FUNCTION "Consensi Linea" : VOID
TITLE =Gestione consensi linea pallet
AUTHOR : MassimoZ
FAMILY : NovaSrl
VERSION : 0.1

BEGIN
NETWORK
TITLE ======== Consensi Vari =======



NETWORK
TITLE =Forzatura dell'Override Limite Max 100%
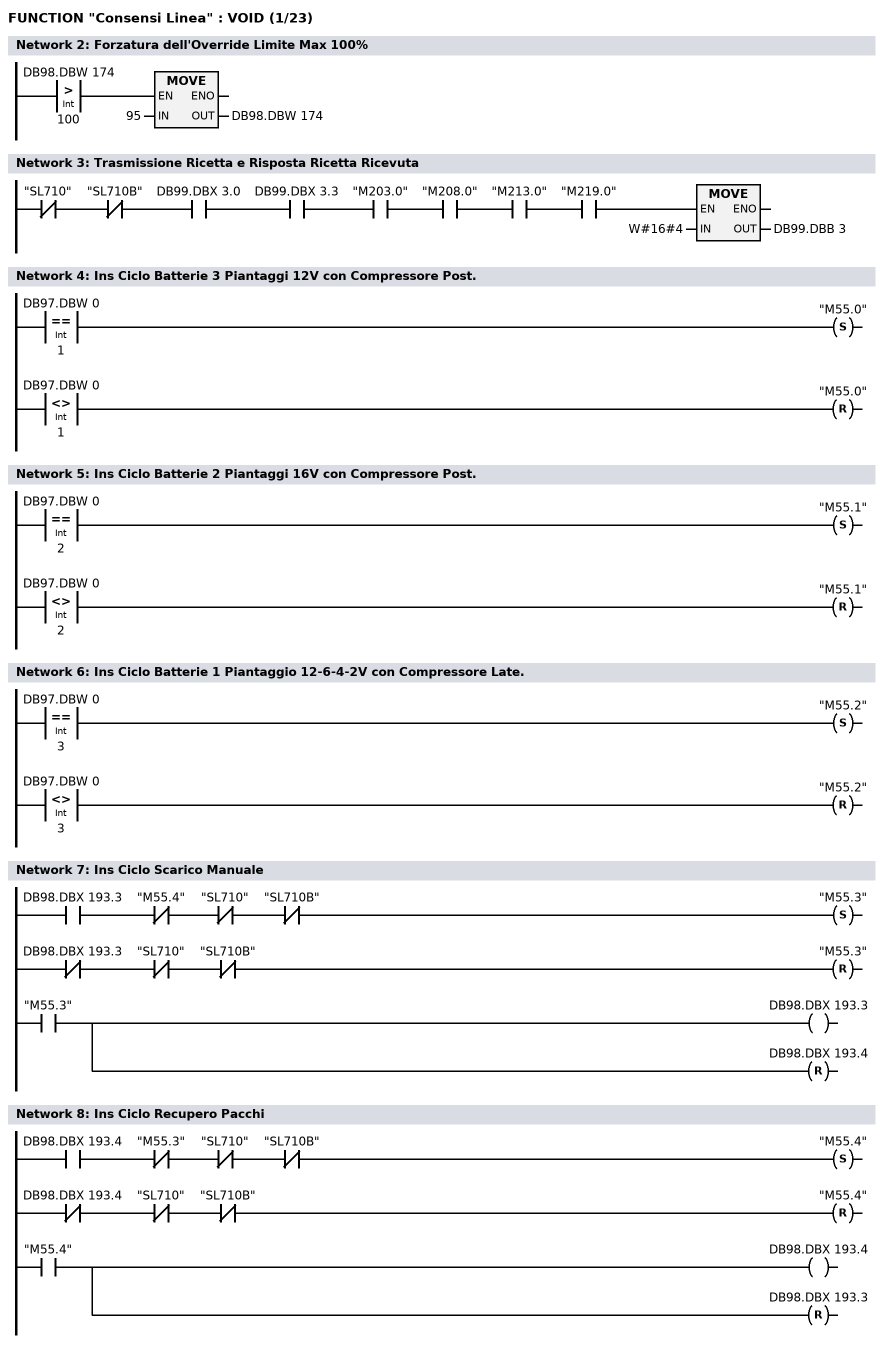
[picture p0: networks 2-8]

      U(    ;
      L     DB98.DBW  174;
      L     100;
      >I    ;
      )     ;
      SPBNB _001;
      L     95;
      T     DB98.DBW  174;
_001: NOP   0;
NETWORK
TITLE =Trasmissione Ricetta e Risposta Ricetta Ricevuta

      UN    "SL710";
      UN    "SL710B";
      U     DB99.DBX    3.0;
      U     DB99.DBX    3.3;
      U     "M203.0";
      U     "M208.0";
      U     "M213.0";
      U     "M219.0";
      SPBNB _002;
      L     W#16#4;
      T     DB99.DBB    3;
_002: NOP   0;
NETWORK
TITLE =Ins Ciclo Batterie 3 Piantaggi 12V con Compressore Post.

      U(    ;
      L     DB97.DBW    0;
      L     1;
      ==I   ;
      )     ;
      S     "M55.0";
      U(    ;
      L     DB97.DBW    0;
      L     1;
      <>I   ;
      )     ;
      R     "M55.0";
      NOP   0;
NETWORK
TITLE =Ins Ciclo Batterie 2 Piantaggi 16V con Compressore Post.

      U(    ;
      L     DB97.DBW    0;
      L     2;
      ==I   ;
      )     ;
      S     "M55.1";
      U(    ;
      L     DB97.DBW    0;
      L     2;
      <>I   ;
      )     ;
      R     "M55.1";
      NOP   0;
NETWORK
TITLE =Ins Ciclo Batterie 1 Piantaggio 12-6-4-2V con Compressore Late.

      U(    ;
      L     DB97.DBW    0;
      L     3;
      ==I   ;
      )     ;
      S     "M55.2";
      U(    ;
      L     DB97.DBW    0;
      L     3;
      <>I   ;
      )     ;
      R     "M55.2";
      NOP   0;
NETWORK
TITLE =Ins Ciclo Scarico Manuale

      U     DB98.DBX  193.3;
      UN    "M55.4";
      UN    "SL710";
      UN    "SL710B";
      S     "M55.3";
      UN    DB98.DBX  193.3;
      UN    "SL710";
      UN    "SL710B";
      R     "M55.3";
      U     "M55.3";
      =     DB98.DBX  193.3;
      R     DB98.DBX  193.4;
NETWORK
TITLE =Ins Ciclo Recupero Pacchi

      U     DB98.DBX  193.4;
      UN    "M55.3";
      UN    "SL710";
      UN    "SL710B";
      S     "M55.4";
      UN    DB98.DBX  193.4;
      UN    "SL710";
      UN    "SL710B";
      R     "M55.4";
      U     "M55.4";
      =     DB98.DBX  193.4;
      R     DB98.DBX  193.3;
NETWORK
TITLE =Visualizzazione a Pannello del Ciclo 3 Piantaggi Inserito
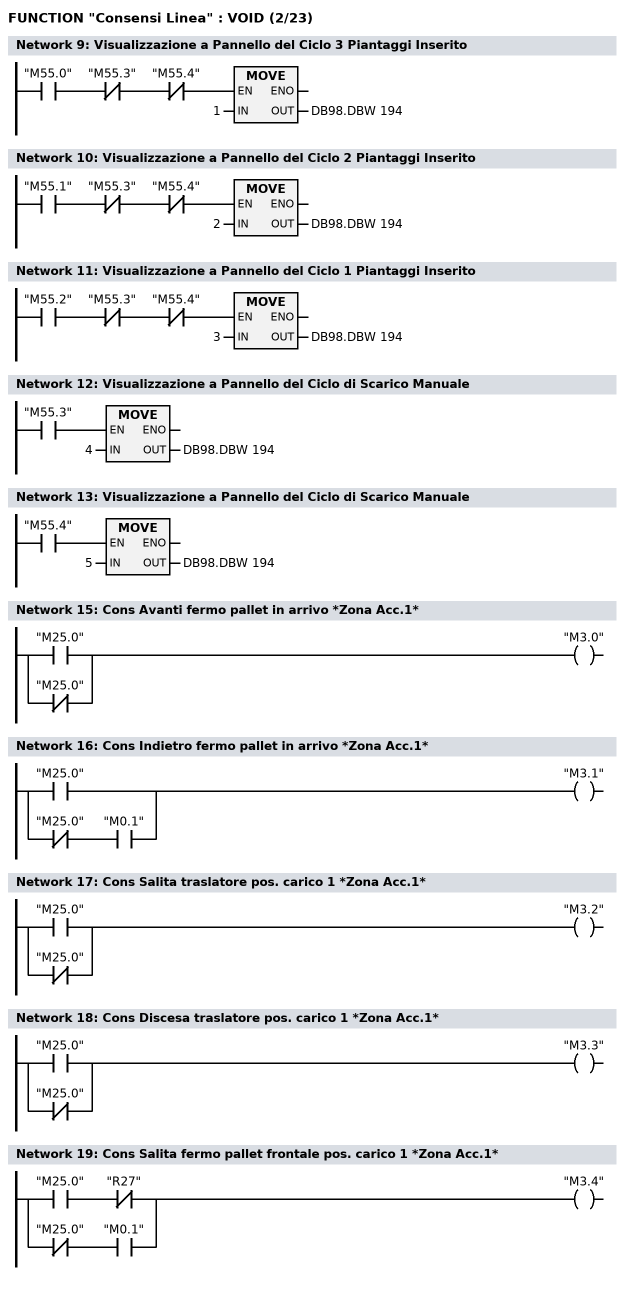
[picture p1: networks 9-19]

      U     "M55.0";
      UN    "M55.3";
      UN    "M55.4";
      SPBNB _003;
      L     1;
      T     DB98.DBW  194;
_003: NOP   0;
NETWORK
TITLE =Visualizzazione a Pannello del Ciclo 2 Piantaggi Inserito

      U     "M55.1";
      UN    "M55.3";
      UN    "M55.4";
      SPBNB _004;
      L     2;
      T     DB98.DBW  194;
_004: NOP   0;
NETWORK
TITLE =Visualizzazione a Pannello del Ciclo 1 Piantaggi Inserito

      U     "M55.2";
      UN    "M55.3";
      UN    "M55.4";
      SPBNB _005;
      L     3;
      T     DB98.DBW  194;
_005: NOP   0;
NETWORK
TITLE =Visualizzazione a Pannello del Ciclo di Scarico Manuale

      U     "M55.3";
      SPBNB _006;
      L     4;
      T     DB98.DBW  194;
_006: NOP   0;
NETWORK
TITLE =Visualizzazione a Pannello del Ciclo di Scarico Manuale

      U     "M55.4";
      SPBNB _007;
      L     5;
      T     DB98.DBW  194;
_007: NOP   0;
NETWORK
TITLE ========= Consensi Zona Accatastatrice 1 =======



NETWORK
TITLE =Cons Avanti fermo pallet in arrivo *Zona Acc.1*

      O     "M25.0";
      ON    "M25.0";
      =     "M3.0";
NETWORK
TITLE =Cons Indietro fermo pallet in arrivo *Zona Acc.1*

      O     "M25.0";
      O     ;
      UN    "M25.0";
      U     "M0.1";
      =     "M3.1";
NETWORK
TITLE =Cons Salita traslatore pos. carico 1 *Zona Acc.1*

      O     "M25.0";
      ON    "M25.0";
      =     "M3.2";
NETWORK
TITLE =Cons Discesa traslatore pos. carico 1 *Zona Acc.1*

      O     "M25.0";
      ON    "M25.0";
      =     "M3.3";
NETWORK
TITLE =Cons Salita fermo pallet frontale pos. carico 1 *Zona Acc.1*

      U     "M25.0";
      UN    "R27";
      O     ;
      UN    "M25.0";
      U     "M0.1";
      =     "M3.4";
NETWORK
TITLE =Cons Discesa fermo pallet frontale pos. carico 1 *Zona Acc.1*
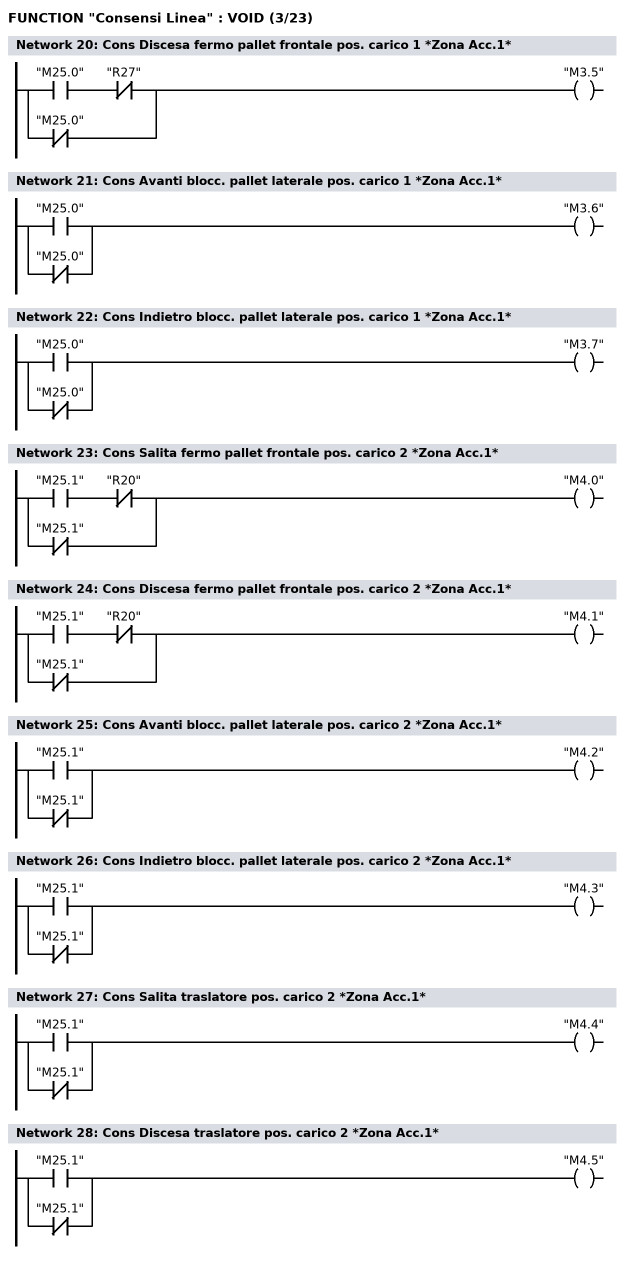
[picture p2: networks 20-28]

      U     "M25.0";
      UN    "R27";
      ON    "M25.0";
      =     "M3.5";
NETWORK
TITLE =Cons Avanti blocc. pallet laterale pos. carico 1 *Zona Acc.1*

      O     "M25.0";
      ON    "M25.0";
      =     "M3.6";
NETWORK
TITLE =Cons Indietro blocc. pallet laterale pos. carico 1 *Zona Acc.1*

      O     "M25.0";
      ON    "M25.0";
      =     "M3.7";
NETWORK
TITLE =Cons Salita fermo pallet frontale pos. carico 2 *Zona Acc.1*

      U     "M25.1";
      UN    "R20";
      ON    "M25.1";
      =     "M4.0";
NETWORK
TITLE =Cons Discesa fermo pallet frontale pos. carico 2 *Zona Acc.1*

      U     "M25.1";
      UN    "R20";
      ON    "M25.1";
      =     "M4.1";
NETWORK
TITLE =Cons Avanti blocc. pallet laterale pos. carico 2 *Zona Acc.1*

      O     "M25.1";
      ON    "M25.1";
      =     "M4.2";
NETWORK
TITLE =Cons Indietro blocc. pallet laterale pos. carico 2 *Zona Acc.1*

      O     "M25.1";
      ON    "M25.1";
      =     "M4.3";
NETWORK
TITLE =Cons Salita traslatore pos. carico 2 *Zona Acc.1*

      O     "M25.1";
      ON    "M25.1";
      =     "M4.4";
NETWORK
TITLE =Cons Discesa traslatore pos. carico 2 *Zona Acc.1*

      O     "M25.1";
      ON    "M25.1";
      =     "M4.5";
NETWORK
TITLE =Cons Salita fermo pallet in uscita *Zona Acc.1*
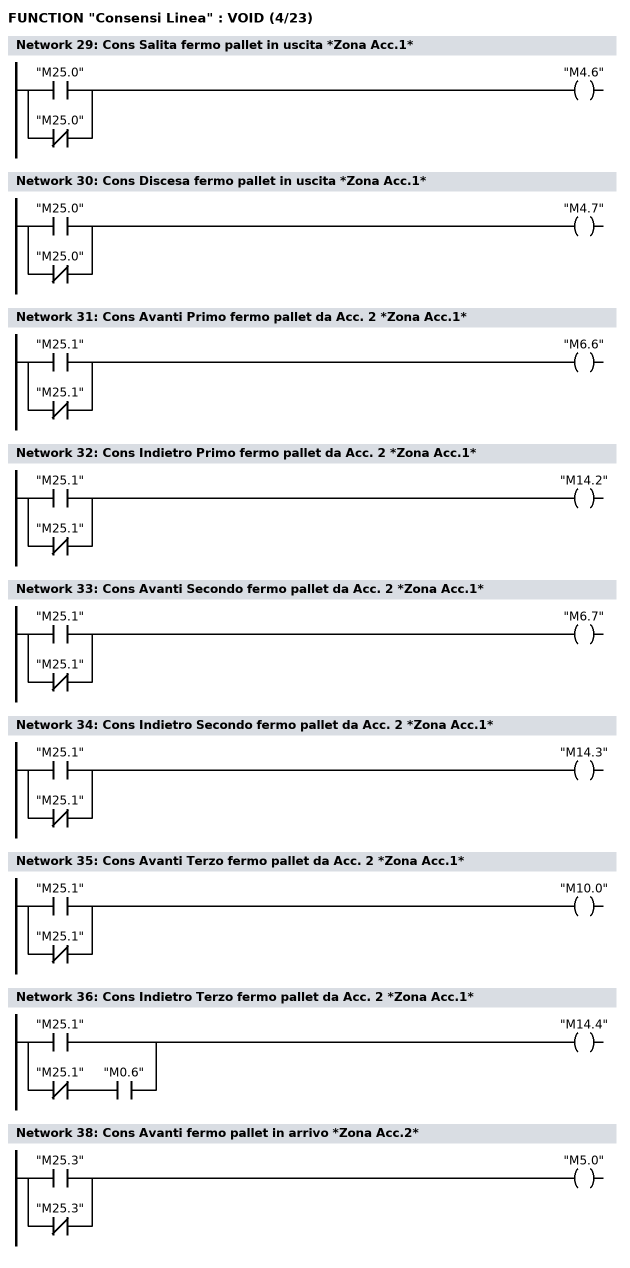
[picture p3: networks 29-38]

      O     "M25.0";
      ON    "M25.0";
      =     "M4.6";
NETWORK
TITLE =Cons Discesa fermo pallet in uscita *Zona Acc.1*

      O     "M25.0";
      ON    "M25.0";
      =     "M4.7";
NETWORK
TITLE =Cons Avanti Primo fermo pallet da Acc. 2 *Zona Acc.1*

      O     "M25.1";
      ON    "M25.1";
      =     "M6.6";
NETWORK
TITLE =Cons Indietro Primo fermo pallet da Acc. 2 *Zona Acc.1*

      O     "M25.1";
      ON    "M25.1";
      =     "M14.2";
NETWORK
TITLE =Cons Avanti Secondo fermo pallet da Acc. 2 *Zona Acc.1*

      O     "M25.1";
      ON    "M25.1";
      =     "M6.7";
NETWORK
TITLE =Cons Indietro Secondo fermo pallet da Acc. 2 *Zona Acc.1*

      O     "M25.1";
      ON    "M25.1";
      =     "M14.3";
NETWORK
TITLE =Cons Avanti Terzo fermo pallet da Acc. 2 *Zona Acc.1*

      O     "M25.1";
      ON    "M25.1";
      =     "M10.0";
NETWORK
TITLE =Cons Indietro Terzo fermo pallet da Acc. 2 *Zona Acc.1*

      O     "M25.1";
      O     ;
      UN    "M25.1";
      U     "M0.6";
      =     "M14.4";
NETWORK
TITLE ========= Consensi Zona Accatastatrice 2 =======



NETWORK
TITLE =Cons Avanti fermo pallet in arrivo *Zona Acc.2*

      O     "M25.3";
      ON    "M25.3";
      =     "M5.0";
NETWORK
TITLE =Cons Indietro fermo pallet in arrivo *Zona Acc.2*
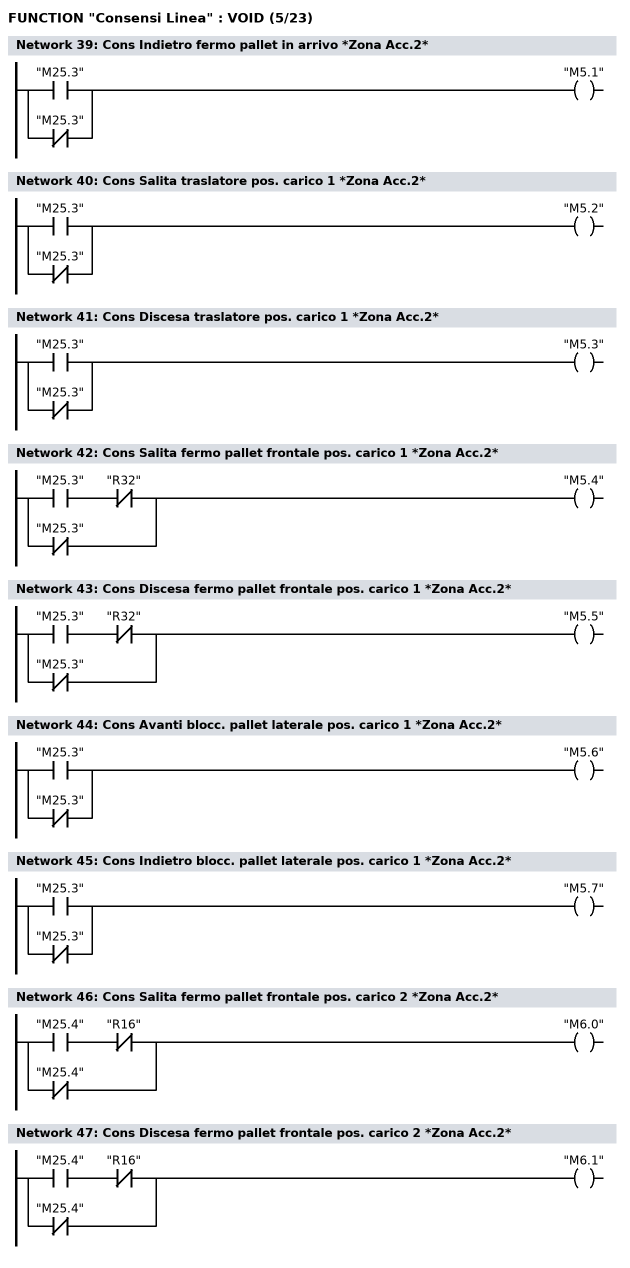
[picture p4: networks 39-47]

      O     "M25.3";
      ON    "M25.3";
      =     "M5.1";
NETWORK
TITLE =Cons Salita traslatore pos. carico 1 *Zona Acc.2*

      O     "M25.3";
      ON    "M25.3";
      =     "M5.2";
NETWORK
TITLE =Cons Discesa traslatore pos. carico 1 *Zona Acc.2*

      O     "M25.3";
      ON    "M25.3";
      =     "M5.3";
NETWORK
TITLE =Cons Salita fermo pallet frontale pos. carico 1 *Zona Acc.2*

      U     "M25.3";
      UN    "R32";
      ON    "M25.3";
      =     "M5.4";
NETWORK
TITLE =Cons Discesa fermo pallet frontale pos. carico 1 *Zona Acc.2*

      U     "M25.3";
      UN    "R32";
      ON    "M25.3";
      =     "M5.5";
NETWORK
TITLE =Cons Avanti blocc. pallet laterale pos. carico 1 *Zona Acc.2*

      O     "M25.3";
      ON    "M25.3";
      =     "M5.6";
NETWORK
TITLE =Cons Indietro blocc. pallet laterale pos. carico 1 *Zona Acc.2*

      O     "M25.3";
      ON    "M25.3";
      =     "M5.7";
NETWORK
TITLE =Cons Salita fermo pallet frontale pos. carico 2 *Zona Acc.2*

      U     "M25.4";
      UN    "R16";
      ON    "M25.4";
      =     "M6.0";
NETWORK
TITLE =Cons Discesa fermo pallet frontale pos. carico 2 *Zona Acc.2*

      U     "M25.4";
      UN    "R16";
      ON    "M25.4";
      =     "M6.1";
NETWORK
TITLE =Cons Avanti blocc. pallet laterale pos. carico 2 *Zona Acc.2*
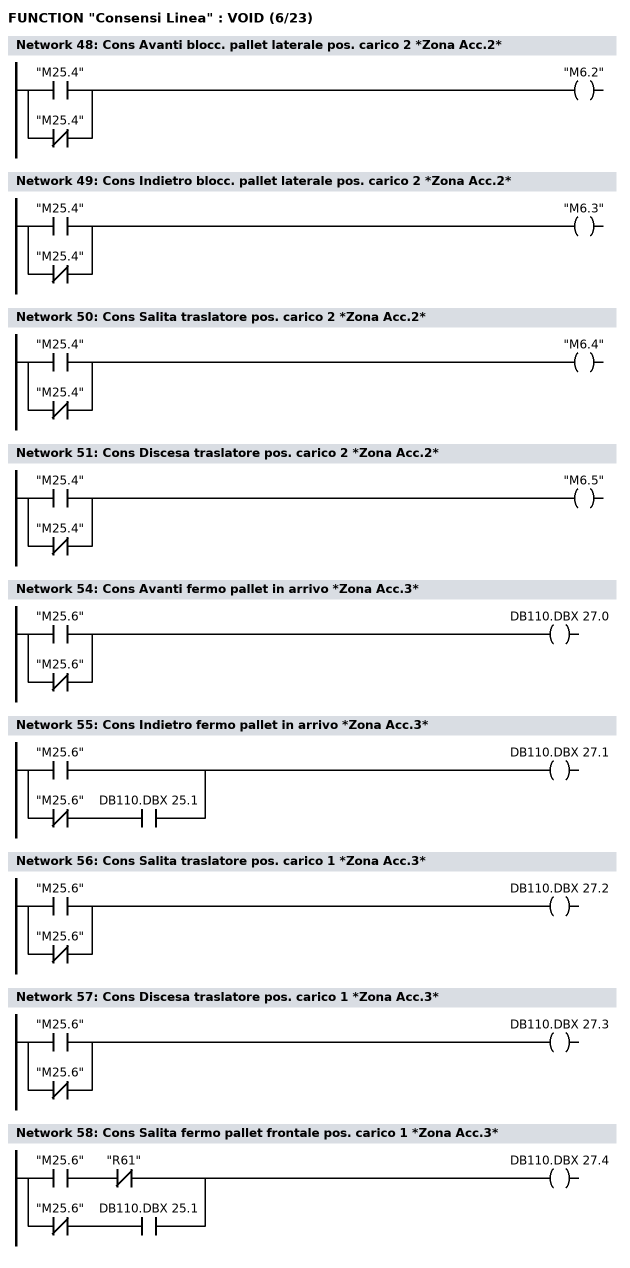
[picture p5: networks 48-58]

      O     "M25.4";
      ON    "M25.4";
      =     "M6.2";
NETWORK
TITLE =Cons Indietro blocc. pallet laterale pos. carico 2 *Zona Acc.2*

      O     "M25.4";
      ON    "M25.4";
      =     "M6.3";
NETWORK
TITLE =Cons Salita traslatore pos. carico 2 *Zona Acc.2*

      O     "M25.4";
      ON    "M25.4";
      =     "M6.4";
NETWORK
TITLE =Cons Discesa traslatore pos. carico 2 *Zona Acc.2*

      O     "M25.4";
      ON    "M25.4";
      =     "M6.5";
NETWORK
TITLE =

NETWORK
TITLE ========= Consensi Zona Accatastatrice 3 =======

NETWORK
TITLE =Cons Avanti fermo pallet in arrivo *Zona Acc.3*

      O     "M25.6";
      ON    "M25.6";
      =     DB110.DBX   27.0;
NETWORK
TITLE =Cons Indietro fermo pallet in arrivo *Zona Acc.3*

      O     "M25.6";
      O     ;
      UN    "M25.6";
      U     DB110.DBX   25.1;
      =     DB110.DBX   27.1;
NETWORK
TITLE =Cons Salita traslatore pos. carico 1 *Zona Acc.3*

      O     "M25.6";
      ON    "M25.6";
      =     DB110.DBX   27.2;
NETWORK
TITLE =Cons Discesa traslatore pos. carico 1 *Zona Acc.3*

      O     "M25.6";
      ON    "M25.6";
      =     DB110.DBX   27.3;
NETWORK
TITLE =Cons Salita fermo pallet frontale pos. carico 1 *Zona Acc.3*

      U     "M25.6";
      UN    "R61";
      O     ;
      UN    "M25.6";
      U     DB110.DBX   25.1;
      =     DB110.DBX   27.4;
NETWORK
TITLE =Cons Discesa fermo pallet frontale pos. carico 1 *Zona Acc.3*
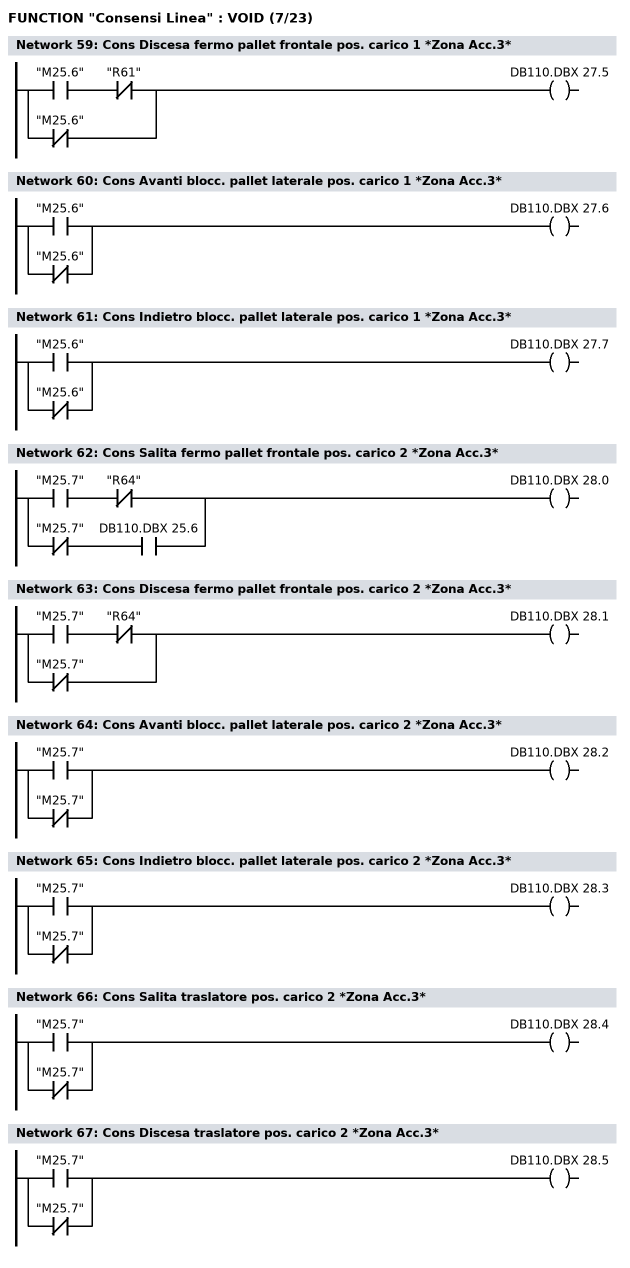
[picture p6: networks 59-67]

      U     "M25.6";
      UN    "R61";
      ON    "M25.6";
      =     DB110.DBX   27.5;
NETWORK
TITLE =Cons Avanti blocc. pallet laterale pos. carico 1 *Zona Acc.3*

      O     "M25.6";
      ON    "M25.6";
      =     DB110.DBX   27.6;
NETWORK
TITLE =Cons Indietro blocc. pallet laterale pos. carico 1 *Zona Acc.3*

      O     "M25.6";
      ON    "M25.6";
      =     DB110.DBX   27.7;
NETWORK
TITLE =Cons Salita fermo pallet frontale pos. carico 2 *Zona Acc.3*

      U     "M25.7";
      UN    "R64";
      O     ;
      UN    "M25.7";
      U     DB110.DBX   25.6;
      =     DB110.DBX   28.0;
NETWORK
TITLE =Cons Discesa fermo pallet frontale pos. carico 2 *Zona Acc.3*

      U     "M25.7";
      UN    "R64";
      ON    "M25.7";
      =     DB110.DBX   28.1;
NETWORK
TITLE =Cons Avanti blocc. pallet laterale pos. carico 2 *Zona Acc.3*

      O     "M25.7";
      ON    "M25.7";
      =     DB110.DBX   28.2;
NETWORK
TITLE =Cons Indietro blocc. pallet laterale pos. carico 2 *Zona Acc.3*

      O     "M25.7";
      ON    "M25.7";
      =     DB110.DBX   28.3;
NETWORK
TITLE =Cons Salita traslatore pos. carico 2 *Zona Acc.3*

      O     "M25.7";
      ON    "M25.7";
      =     DB110.DBX   28.4;
NETWORK
TITLE =Cons Discesa traslatore pos. carico 2 *Zona Acc.3*

      O     "M25.7";
      ON    "M25.7";
      =     DB110.DBX   28.5;
NETWORK
TITLE =Cons Salita fermo pallet in uscita *Zona Acc.3*
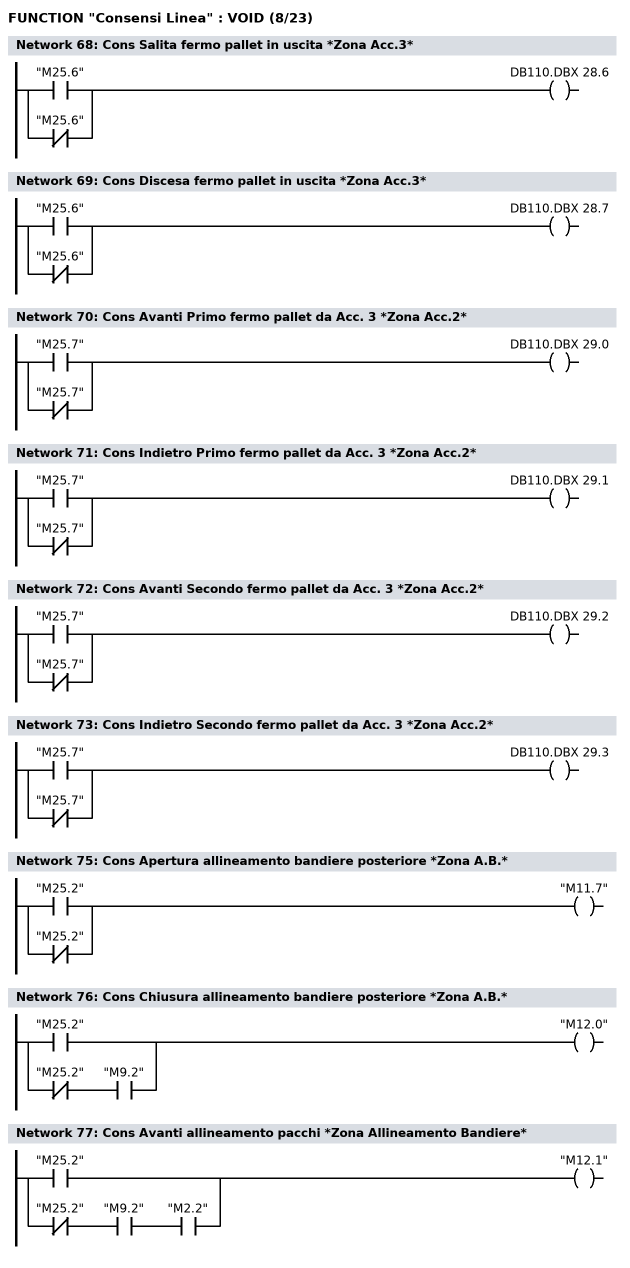
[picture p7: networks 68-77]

      O     "M25.6";
      ON    "M25.6";
      =     DB110.DBX   28.6;
NETWORK
TITLE =Cons Discesa fermo pallet in uscita *Zona Acc.3*

      O     "M25.6";
      ON    "M25.6";
      =     DB110.DBX   28.7;
NETWORK
TITLE =Cons Avanti Primo fermo pallet da Acc. 3 *Zona Acc.2*

      O     "M25.7";
      ON    "M25.7";
      =     DB110.DBX   29.0;
NETWORK
TITLE =Cons Indietro Primo fermo pallet da Acc. 3 *Zona Acc.2*

      O     "M25.7";
      ON    "M25.7";
      =     DB110.DBX   29.1;
NETWORK
TITLE =Cons Avanti Secondo fermo pallet da Acc. 3 *Zona Acc.2*

      O     "M25.7";
      ON    "M25.7";
      =     DB110.DBX   29.2;
NETWORK
TITLE =Cons Indietro Secondo fermo pallet da Acc. 3 *Zona Acc.2*

      O     "M25.7";
      ON    "M25.7";
      =     DB110.DBX   29.3;
NETWORK
TITLE ======== Consensi Zona Allineamento Bandiere =======



NETWORK
TITLE =Cons Apertura allineamento bandiere posteriore *Zona A.B.*

      O     "M25.2";
      ON    "M25.2";
      =     "M11.7";
NETWORK
TITLE =Cons Chiusura allineamento bandiere posteriore *Zona A.B.*

      O     "M25.2";
      O     ;
      UN    "M25.2";
      U     "M9.2";
      =     "M12.0";
NETWORK
TITLE =Cons Avanti allineamento pacchi *Zona Allineamento Bandiere*

      O     "M25.2";
      O     ;
      UN    "M25.2";
      U     "M9.2";
      U     "M2.2";
      =     "M12.1";
NETWORK
TITLE =Cons Indietro allineamento pacchi *Zona Allineamento Bandiere*
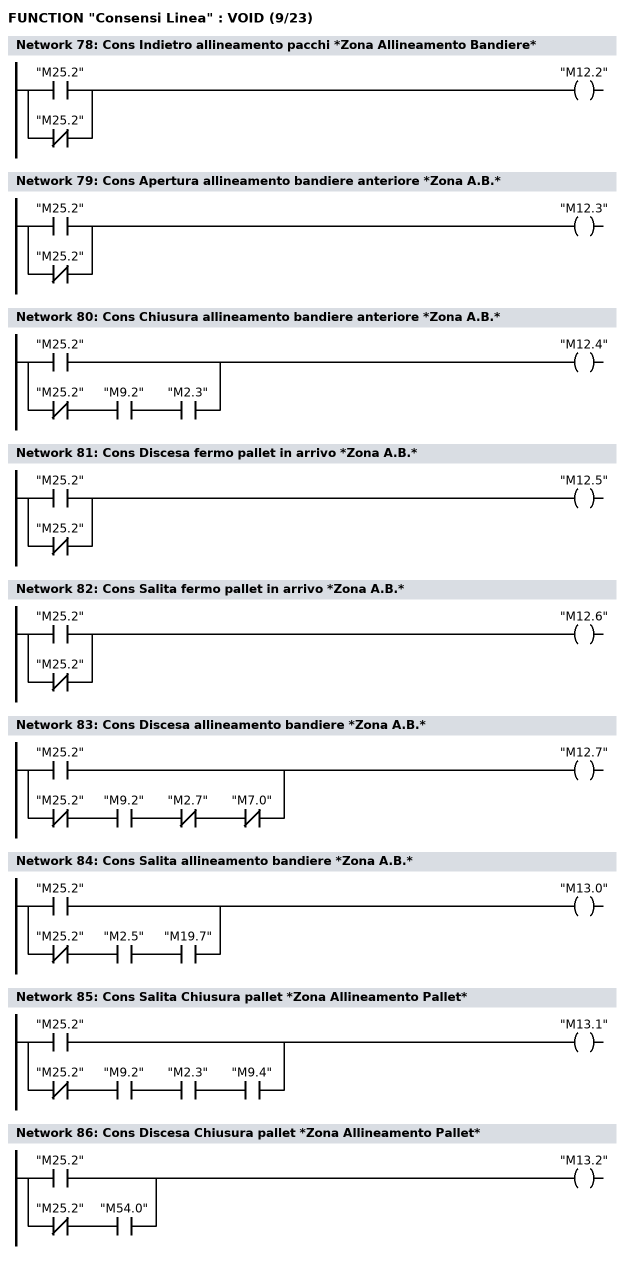
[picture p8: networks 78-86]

      O     "M25.2";
      ON    "M25.2";
      =     "M12.2";
NETWORK
TITLE =Cons Apertura allineamento bandiere anteriore *Zona A.B.*

      O     "M25.2";
      ON    "M25.2";
      =     "M12.3";
NETWORK
TITLE =Cons Chiusura allineamento bandiere anteriore *Zona A.B.*

      O     "M25.2";
      O     ;
      UN    "M25.2";
      U     "M9.2";
      U     "M2.3";
      =     "M12.4";
NETWORK
TITLE =Cons Discesa fermo pallet in arrivo *Zona A.B.*

      O     "M25.2";
      ON    "M25.2";
      =     "M12.5";
NETWORK
TITLE =Cons Salita fermo pallet in arrivo *Zona A.B.*

      O     "M25.2";
      ON    "M25.2";
      =     "M12.6";
NETWORK
TITLE =Cons Discesa allineamento bandiere *Zona A.B.*

      O     "M25.2";
      O     ;
      UN    "M25.2";
      U     "M9.2";
      UN    "M2.7";
      UN    "M7.0";
      =     "M12.7";
NETWORK
TITLE =Cons Salita allineamento bandiere *Zona A.B.*

      O     "M25.2";
      O     ;
      UN    "M25.2";
      U     "M2.5";
      U     "M19.7";
      =     "M13.0";
NETWORK
TITLE =Cons Salita Chiusura pallet *Zona Allineamento Pallet*

      O     "M25.2";
      O     ;
      UN    "M25.2";
      U     "M9.2";
      U     "M2.3";
      U     "M9.4";
      =     "M13.1";
NETWORK
TITLE =Cons Discesa Chiusura pallet *Zona Allineamento Pallet*

      O     "M25.2";
      O     ;
      UN    "M25.2";
      U     "M54.0";
      =     "M13.2";
NETWORK
TITLE =Cons Avanti Chiusura pallet *Zona Allineamento Pallet*
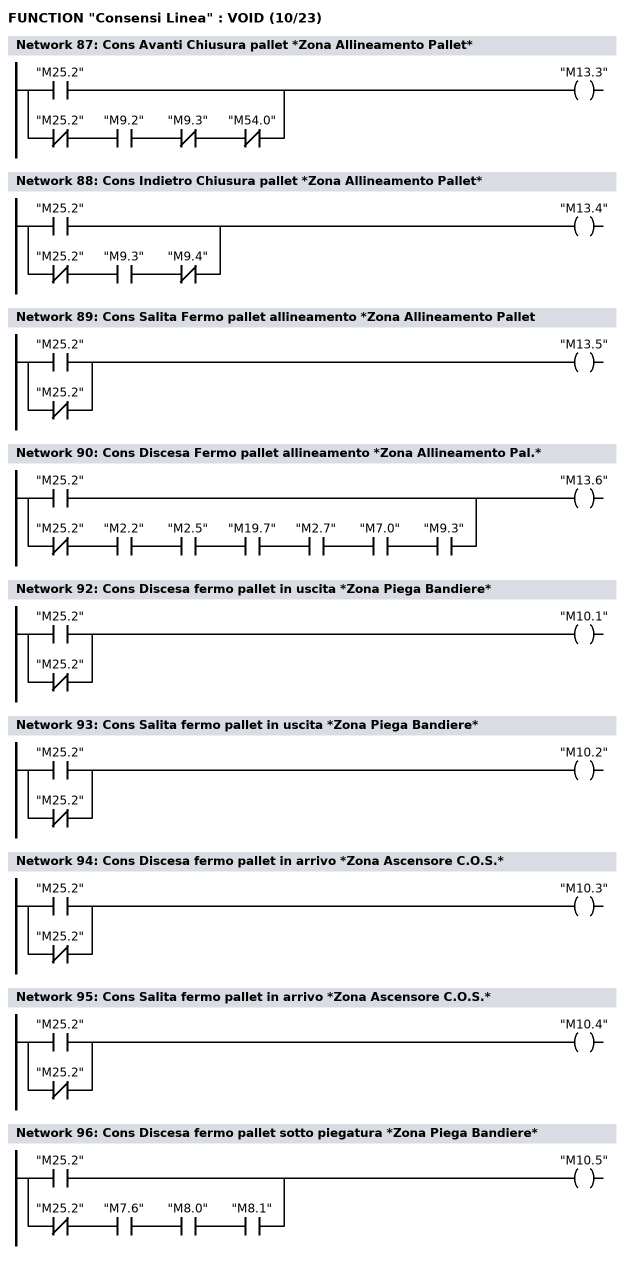
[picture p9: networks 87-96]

      O     "M25.2";
      O     ;
      UN    "M25.2";
      U     "M9.2";
      UN    "M9.3";
      UN    "M54.0";
      =     "M13.3";
NETWORK
TITLE =Cons Indietro Chiusura pallet *Zona Allineamento Pallet*

      O     "M25.2";
      O     ;
      UN    "M25.2";
      U     "M9.3";
      UN    "M9.4";
      =     "M13.4";
NETWORK
TITLE =Cons Salita Fermo pallet allineamento *Zona Allineamento Pallet

      O     "M25.2";
      ON    "M25.2";
      =     "M13.5";
NETWORK
TITLE =Cons Discesa Fermo pallet allineamento *Zona Allineamento Pal.*

      O     "M25.2";
      O     ;
      UN    "M25.2";
      U     "M2.2";
      U     "M2.5";
      U     "M19.7";
      U     "M2.7";
      U     "M7.0";
      U     "M9.3";
      =     "M13.6";
NETWORK
TITLE ======== Consensi Zona Piegatura Bandiere =======



NETWORK
TITLE =Cons Discesa fermo pallet in uscita *Zona Piega Bandiere*

      O     "M25.2";
      ON    "M25.2";
      =     "M10.1";
NETWORK
TITLE =Cons Salita fermo pallet in uscita *Zona Piega Bandiere*

      O     "M25.2";
      ON    "M25.2";
      =     "M10.2";
NETWORK
TITLE =Cons Discesa fermo pallet in arrivo *Zona Ascensore C.O.S.*

      O     "M25.2";
      ON    "M25.2";
      =     "M10.3";
NETWORK
TITLE =Cons Salita fermo pallet in arrivo *Zona Ascensore C.O.S.*

      O     "M25.2";
      ON    "M25.2";
      =     "M10.4";
NETWORK
TITLE =Cons Discesa fermo pallet sotto piegatura *Zona Piega Bandiere*

      O     "M25.2";
      O     ;
      UN    "M25.2";
      U     "M7.6";
      U     "M8.0";
      U     "M8.1";
      =     "M10.5";
NETWORK
TITLE =Cons Salita fermo pallet sotto piegatura *Zona Piega Bandiere*
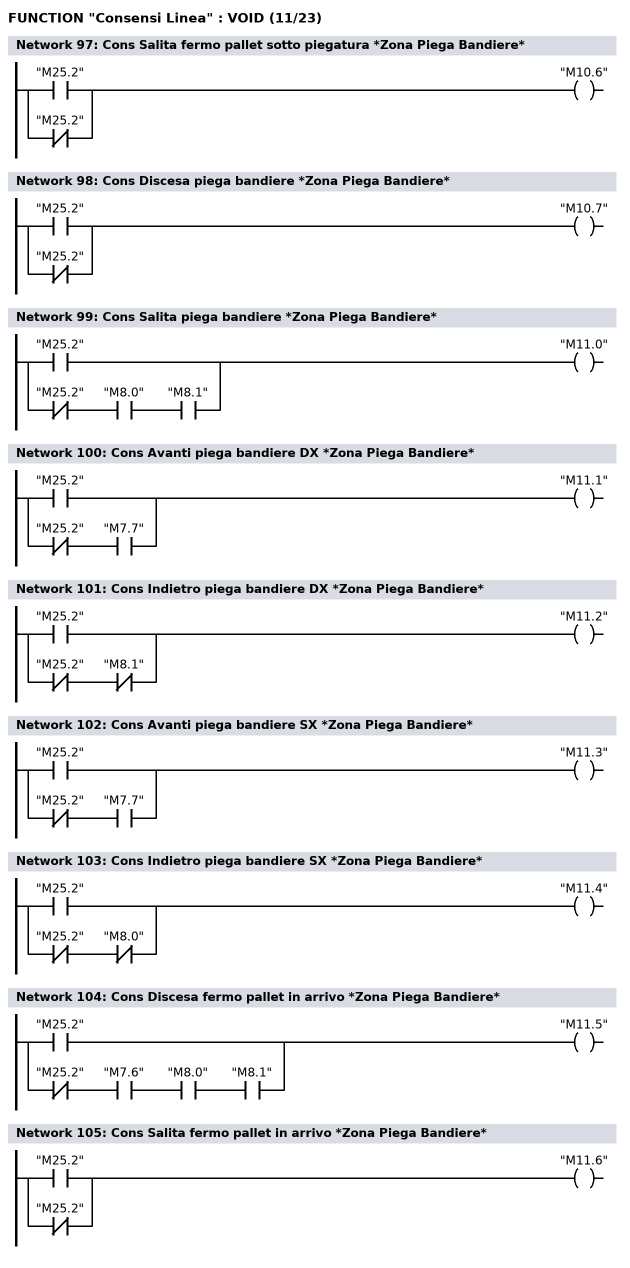
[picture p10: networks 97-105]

      O     "M25.2";
      ON    "M25.2";
      =     "M10.6";
NETWORK
TITLE =Cons Discesa piega bandiere *Zona Piega Bandiere*

      O     "M25.2";
      ON    "M25.2";
      =     "M10.7";
NETWORK
TITLE =Cons Salita piega bandiere *Zona Piega Bandiere*

      O     "M25.2";
      O     ;
      UN    "M25.2";
      U     "M8.0";
      U     "M8.1";
      =     "M11.0";
NETWORK
TITLE =Cons Avanti piega bandiere DX *Zona Piega Bandiere*

      O     "M25.2";
      O     ;
      UN    "M25.2";
      U     "M7.7";
      =     "M11.1";
NETWORK
TITLE =Cons Indietro piega bandiere DX *Zona Piega Bandiere*

      O     "M25.2";
      O     ;
      UN    "M25.2";
      UN    "M8.1";
      =     "M11.2";
NETWORK
TITLE =Cons Avanti piega bandiere SX *Zona Piega Bandiere*

      O     "M25.2";
      O     ;
      UN    "M25.2";
      U     "M7.7";
      =     "M11.3";
NETWORK
TITLE =Cons Indietro piega bandiere SX *Zona Piega Bandiere*

      O     "M25.2";
      O     ;
      UN    "M25.2";
      UN    "M8.0";
      =     "M11.4";
NETWORK
TITLE =Cons Discesa fermo pallet in arrivo *Zona Piega Bandiere*

      O     "M25.2";
      O     ;
      UN    "M25.2";
      U     "M7.6";
      U     "M8.0";
      U     "M8.1";
      =     "M11.5";
NETWORK
TITLE =Cons Salita fermo pallet in arrivo *Zona Piega Bandiere*

      O     "M25.2";
      ON    "M25.2";
      =     "M11.6";
NETWORK
TITLE =Cons Salita Fermo Pallet Anteriore su Ascensore C.O.S.
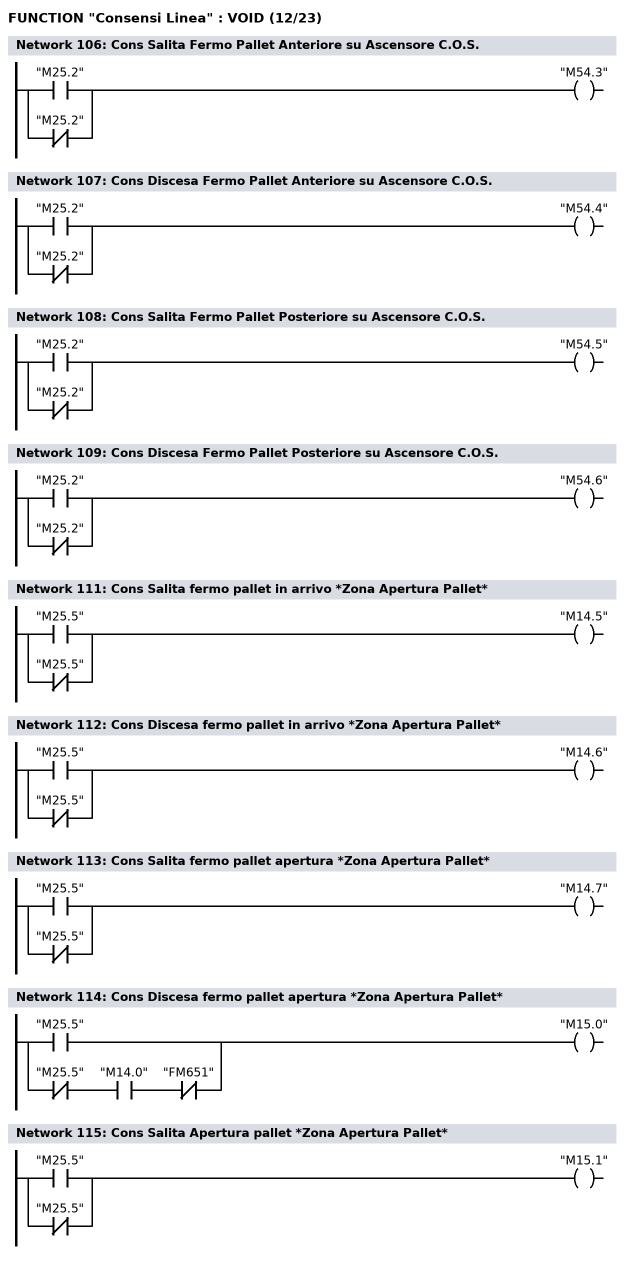
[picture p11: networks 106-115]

      O     "M25.2";
      ON    "M25.2";
      =     "M54.3";
NETWORK
TITLE =Cons Discesa Fermo Pallet Anteriore su Ascensore C.O.S.

      O     "M25.2";
      ON    "M25.2";
      =     "M54.4";
NETWORK
TITLE =Cons Salita Fermo Pallet Posteriore su Ascensore C.O.S.

      O     "M25.2";
      ON    "M25.2";
      =     "M54.5";
NETWORK
TITLE =Cons Discesa Fermo Pallet Posteriore su Ascensore C.O.S.

      O     "M25.2";
      ON    "M25.2";
      =     "M54.6";
NETWORK
TITLE ========= Consensi Zona Apertura Pallet =======



NETWORK
TITLE =Cons Salita fermo pallet in arrivo *Zona Apertura Pallet*

      O     "M25.5";
      ON    "M25.5";
      =     "M14.5";
NETWORK
TITLE =Cons Discesa fermo pallet in arrivo *Zona Apertura Pallet*

      O     "M25.5";
      ON    "M25.5";
      =     "M14.6";
NETWORK
TITLE =Cons Salita fermo pallet apertura *Zona Apertura Pallet*

      O     "M25.5";
      ON    "M25.5";
      =     "M14.7";
NETWORK
TITLE =Cons Discesa fermo pallet apertura *Zona Apertura Pallet*

      O     "M25.5";
      O     ;
      UN    "M25.5";
      U     "M14.0";
      UN    "FM651";
      =     "M15.0";
NETWORK
TITLE =Cons Salita Apertura pallet *Zona Apertura Pallet*

      O     "M25.5";
      ON    "M25.5";
      =     "M15.1";
NETWORK
TITLE =Cons Discesa Apertura pallet *Zona Apertura Pallet*
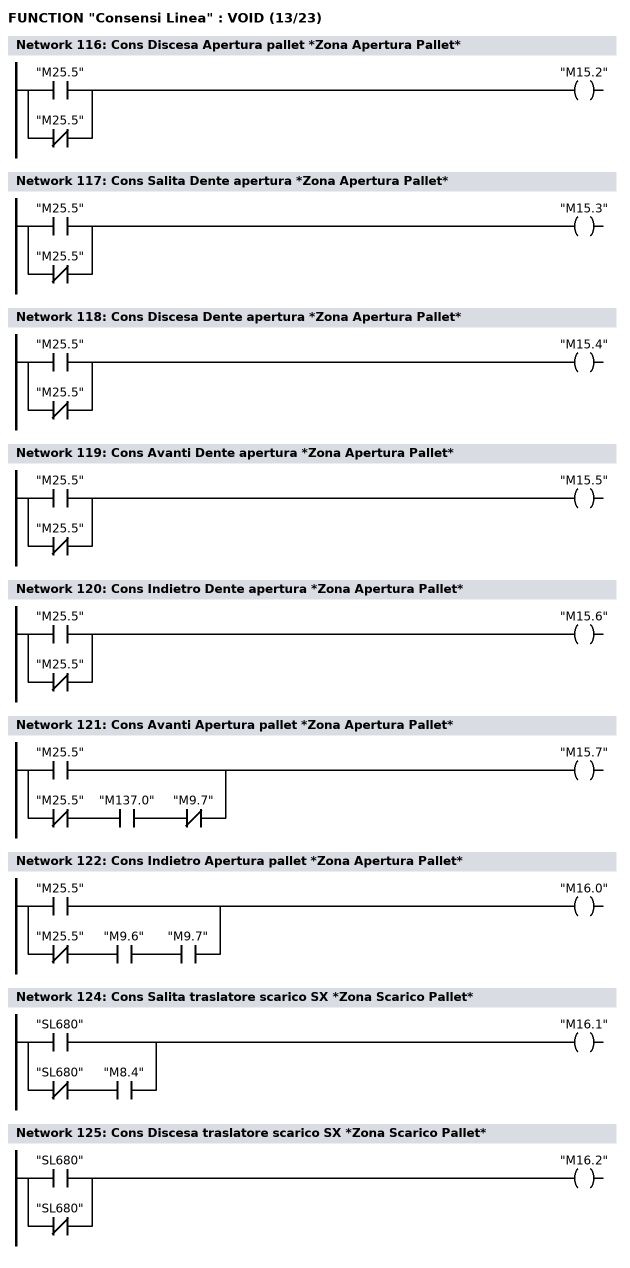
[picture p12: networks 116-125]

      O     "M25.5";
      ON    "M25.5";
      =     "M15.2";
NETWORK
TITLE =Cons Salita Dente apertura *Zona Apertura Pallet*

      O     "M25.5";
      ON    "M25.5";
      =     "M15.3";
NETWORK
TITLE =Cons Discesa Dente apertura *Zona Apertura Pallet*

      O     "M25.5";
      ON    "M25.5";
      =     "M15.4";
NETWORK
TITLE =Cons Avanti Dente apertura *Zona Apertura Pallet*

      O     "M25.5";
      ON    "M25.5";
      =     "M15.5";
NETWORK
TITLE =Cons Indietro Dente apertura *Zona Apertura Pallet*

      O     "M25.5";
      ON    "M25.5";
      =     "M15.6";
NETWORK
TITLE =Cons Avanti Apertura pallet *Zona Apertura Pallet*

      O     "M25.5";
      O     ;
      UN    "M25.5";
      U     "M137.0";
      UN    "M9.7";
      =     "M15.7";
NETWORK
TITLE =Cons Indietro Apertura pallet *Zona Apertura Pallet*

      O     "M25.5";
      O     ;
      UN    "M25.5";
      U     "M9.6";
      U     "M9.7";
      =     "M16.0";
NETWORK
TITLE ======== Consensi Zona Scarico Pallet =======



NETWORK
TITLE =Cons Salita traslatore scarico SX *Zona Scarico Pallet*

      O     "SL680";
      O     ;
      UN    "SL680";
      U     "M8.4";
      =     "M16.1";
NETWORK
TITLE =Cons Discesa traslatore scarico SX *Zona Scarico Pallet*

      O     "SL680";
      ON    "SL680";
      =     "M16.2";
NETWORK
TITLE =Cons Salita traslatore scarico DX *Zona Scarico Pallet*
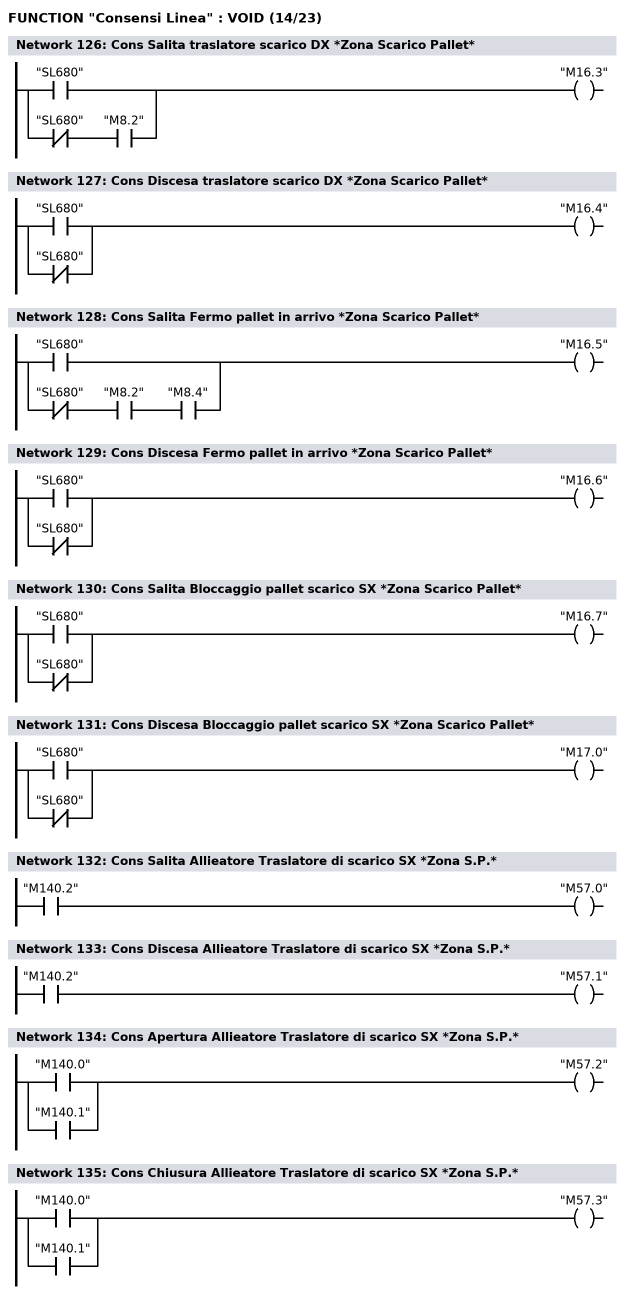
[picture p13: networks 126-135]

      O     "SL680";
      O     ;
      UN    "SL680";
      U     "M8.2";
      =     "M16.3";
NETWORK
TITLE =Cons Discesa traslatore scarico DX *Zona Scarico Pallet*

      O     "SL680";
      ON    "SL680";
      =     "M16.4";
NETWORK
TITLE =Cons Salita Fermo pallet in arrivo *Zona Scarico Pallet*

      O     "SL680";
      O     ;
      UN    "SL680";
      U     "M8.2";
      U     "M8.4";
      =     "M16.5";
NETWORK
TITLE =Cons Discesa Fermo pallet in arrivo *Zona Scarico Pallet*

      O     "SL680";
      ON    "SL680";
      =     "M16.6";
NETWORK
TITLE =Cons Salita Bloccaggio pallet scarico SX *Zona Scarico Pallet*

      O     "SL680";
      ON    "SL680";
      =     "M16.7";
NETWORK
TITLE =Cons Discesa Bloccaggio pallet scarico SX *Zona Scarico Pallet*

      O     "SL680";
      ON    "SL680";
      =     "M17.0";
NETWORK
TITLE =Cons Salita Allieatore Traslatore di scarico SX *Zona S.P.*

      U     "M140.2";
      =     "M57.0";
NETWORK
TITLE =Cons Discesa Allieatore Traslatore di scarico SX *Zona S.P.*

      U     "M140.2";
      =     "M57.1";
NETWORK
TITLE =Cons Apertura Allieatore Traslatore di scarico SX *Zona S.P.*

      O     "M140.0";
      O     "M140.1";
      =     "M57.2";
NETWORK
TITLE =Cons Chiusura Allieatore Traslatore di scarico SX *Zona S.P.*

      O     "M140.0";
      O     "M140.1";
      =     "M57.3";
NETWORK
TITLE =Cons Salita Bloccaggio pallet scarico DX *Zona Scarico Pallet*
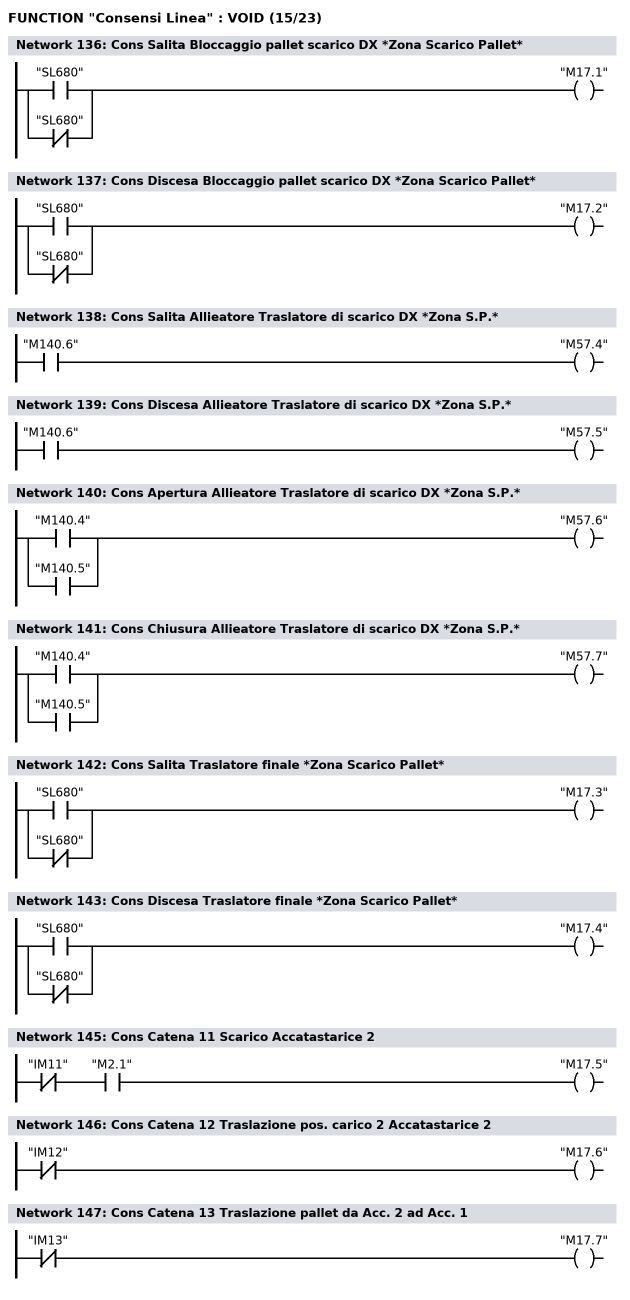
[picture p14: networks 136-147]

      O     "SL680";
      ON    "SL680";
      =     "M17.1";
NETWORK
TITLE =Cons Discesa Bloccaggio pallet scarico DX *Zona Scarico Pallet*

      O     "SL680";
      ON    "SL680";
      =     "M17.2";
NETWORK
TITLE =Cons Salita Allieatore Traslatore di scarico DX *Zona S.P.*

      U     "M140.6";
      =     "M57.4";
NETWORK
TITLE =Cons Discesa Allieatore Traslatore di scarico DX *Zona S.P.*

      U     "M140.6";
      =     "M57.5";
NETWORK
TITLE =Cons Apertura Allieatore Traslatore di scarico DX *Zona S.P.*

      O     "M140.4";
      O     "M140.5";
      =     "M57.6";
NETWORK
TITLE =Cons Chiusura Allieatore Traslatore di scarico DX *Zona S.P.*

      O     "M140.4";
      O     "M140.5";
      =     "M57.7";
NETWORK
TITLE =Cons Salita Traslatore finale *Zona Scarico Pallet*

      O     "SL680";
      ON    "SL680";
      =     "M17.3";
NETWORK
TITLE =Cons Discesa Traslatore finale *Zona Scarico Pallet*

      O     "SL680";
      ON    "SL680";
      =     "M17.4";
NETWORK
TITLE ======== Consenso Catene =======



NETWORK
TITLE =Cons Catena 11 Scarico Accatastarice 2

      UN    "IM11";
      U     "M2.1";
      =     "M17.5";
NETWORK
TITLE =Cons Catena 12 Traslazione pos. carico 2 Accatastarice 2

      UN    "IM12";
      =     "M17.6";
NETWORK
TITLE =Cons Catena 13 Traslazione pallet da Acc. 2 ad Acc. 1

      UN    "IM13";
      =     "M17.7";
NETWORK
TITLE =Cons Catena 14 Traslazione pos. carico 2 Accatastatrice 1
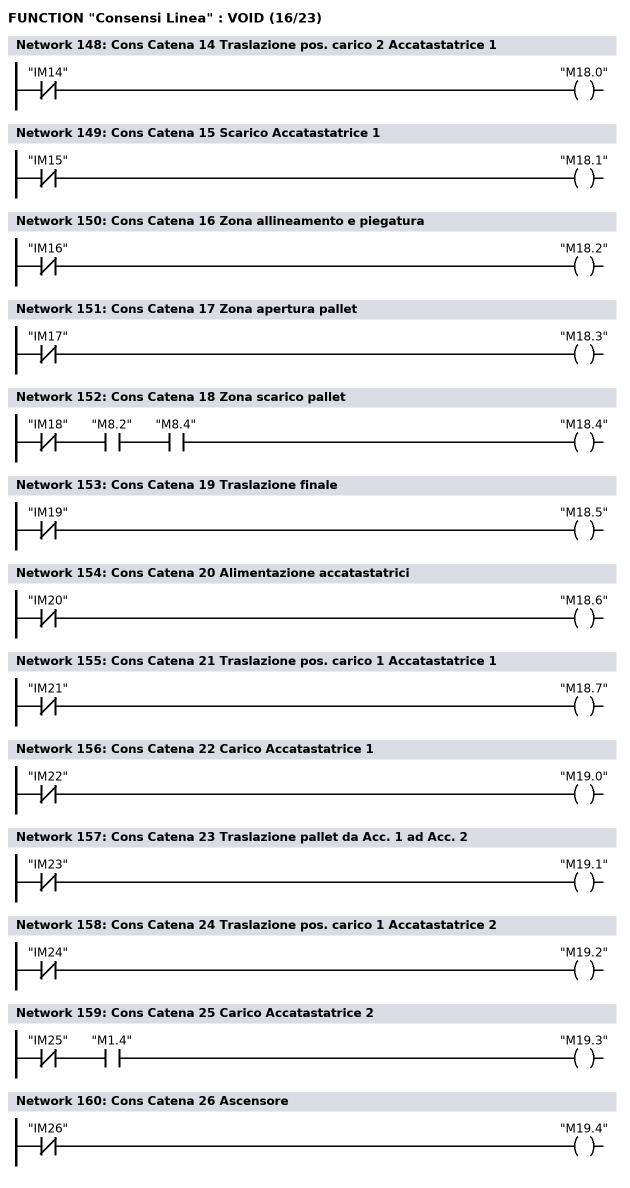
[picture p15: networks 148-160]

      UN    "IM14";
      =     "M18.0";
NETWORK
TITLE =Cons Catena 15 Scarico Accatastatrice 1

      UN    "IM15";
      =     "M18.1";
NETWORK
TITLE =Cons Catena 16 Zona allineamento e piegatura

      UN    "IM16";
      =     "M18.2";
NETWORK
TITLE =Cons Catena 17 Zona apertura pallet

      UN    "IM17";
      =     "M18.3";
NETWORK
TITLE =Cons Catena 18 Zona scarico pallet

      UN    "IM18";
      U     "M8.2";
      U     "M8.4";
      =     "M18.4";
NETWORK
TITLE =Cons Catena 19 Traslazione finale

      UN    "IM19";
      =     "M18.5";
NETWORK
TITLE =Cons Catena 20 Alimentazione accatastatrici

      UN    "IM20";
      =     "M18.6";
NETWORK
TITLE =Cons Catena 21 Traslazione pos. carico 1 Accatastatrice 1

      UN    "IM21";
      =     "M18.7";
NETWORK
TITLE =Cons Catena 22 Carico Accatastatrice 1

      UN    "IM22";
      =     "M19.0";
NETWORK
TITLE =Cons Catena 23 Traslazione pallet da Acc. 1 ad Acc. 2

      UN    "IM23";
      =     "M19.1";
NETWORK
TITLE =Cons Catena 24 Traslazione pos. carico 1 Accatastatrice 2

      UN    "IM24";
      =     "M19.2";
NETWORK
TITLE =Cons Catena 25 Carico Accatastatrice 2

      UN    "IM25";
      U     "M1.4";
      =     "M19.3";
NETWORK
TITLE =Cons Catena 26 Ascensore

      UN    "IM26";
      =     "M19.4";
NETWORK
TITLE =Cons Catena 27 Traslatore scarico DX
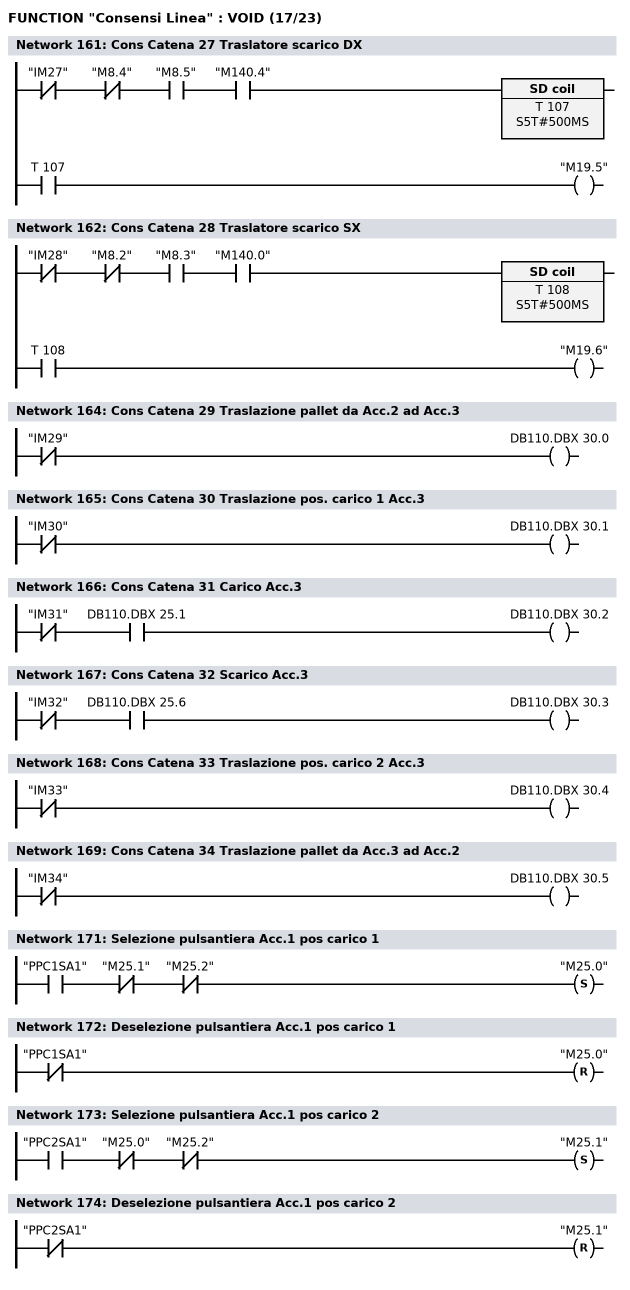
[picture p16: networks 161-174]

      UN    "IM27";
      UN    "M8.4";
      U     "M8.5";
      U     "M140.4";
      L     S5T#500MS;
      SE    T    107;
      NOP   0;
      NOP   0;
      NOP   0;
      U     T    107;
      =     "M19.5";
NETWORK
TITLE =Cons Catena 28 Traslatore scarico SX

      UN    "IM28";
      UN    "M8.2";
      U     "M8.3";
      U     "M140.0";
      L     S5T#500MS;
      SE    T    108;
      NOP   0;
      NOP   0;
      NOP   0;
      U     T    108;
      =     "M19.6";
NETWORK
TITLE =

NETWORK
TITLE =Cons Catena 29 Traslazione pallet da Acc.2 ad Acc.3

      UN    "IM29";
      =     DB110.DBX   30.0;
NETWORK
TITLE =Cons Catena 30 Traslazione pos. carico 1 Acc.3

      UN    "IM30";
      =     DB110.DBX   30.1;
NETWORK
TITLE =Cons Catena 31 Carico Acc.3

      UN    "IM31";
      U     DB110.DBX   25.1;
      =     DB110.DBX   30.2;
NETWORK
TITLE =Cons Catena 32 Scarico Acc.3

      UN    "IM32";
      U     DB110.DBX   25.6;
      =     DB110.DBX   30.3;
NETWORK
TITLE =Cons Catena 33 Traslazione pos. carico 2 Acc.3

      UN    "IM33";
      =     DB110.DBX   30.4;
NETWORK
TITLE =Cons Catena 34 Traslazione pallet da Acc.3 ad Acc.2

      UN    "IM34";
      =     DB110.DBX   30.5;
NETWORK
TITLE ======== Selezioni Pulsantiere =======



NETWORK
TITLE =Selezione pulsantiera Acc.1 pos carico 1

      U     "PPC1SA1";
      UN    "M25.1";
      UN    "M25.2";
      S     "M25.0";
NETWORK
TITLE =Deselezione pulsantiera Acc.1 pos carico 1

      UN    "PPC1SA1";
      R     "M25.0";
NETWORK
TITLE =Selezione pulsantiera Acc.1 pos carico 2

      U     "PPC2SA1";
      UN    "M25.0";
      UN    "M25.2";
      S     "M25.1";
NETWORK
TITLE =Deselezione pulsantiera Acc.1 pos carico 2

      UN    "PPC2SA1";
      R     "M25.1";
NETWORK
TITLE =Selezione pulsantiera zona Allineamento + Piega
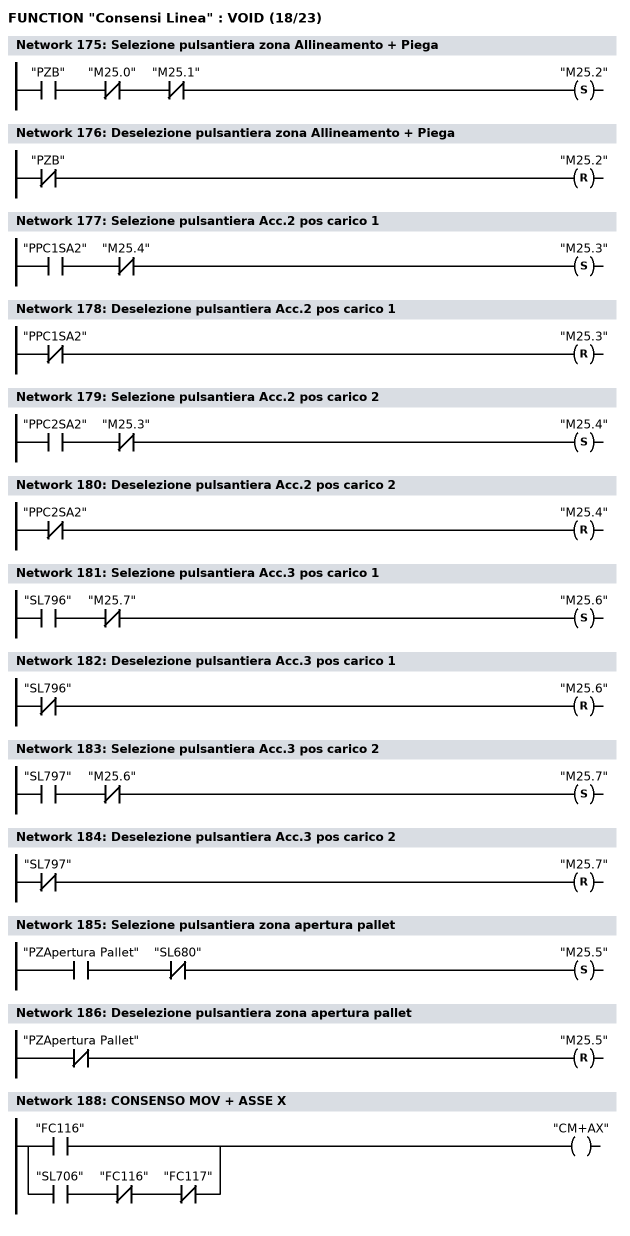
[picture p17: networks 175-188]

      U     "PZB";
      UN    "M25.0";
      UN    "M25.1";
      S     "M25.2";
NETWORK
TITLE =Deselezione pulsantiera zona Allineamento + Piega

      UN    "PZB";
      R     "M25.2";
NETWORK
TITLE =Selezione pulsantiera Acc.2 pos carico 1

      U     "PPC1SA2";
      UN    "M25.4";
      S     "M25.3";
NETWORK
TITLE =Deselezione pulsantiera Acc.2 pos carico 1

      UN    "PPC1SA2";
      R     "M25.3";
NETWORK
TITLE =Selezione pulsantiera Acc.2 pos carico 2

      U     "PPC2SA2";
      UN    "M25.3";
      S     "M25.4";
NETWORK
TITLE =Deselezione pulsantiera Acc.2 pos carico 2

      UN    "PPC2SA2";
      R     "M25.4";
NETWORK
TITLE =Selezione pulsantiera Acc.3 pos carico 1

      U     "SL796";
      UN    "M25.7";
      S     "M25.6";
NETWORK
TITLE =Deselezione pulsantiera Acc.3 pos carico 1

      UN    "SL796";
      R     "M25.6";
NETWORK
TITLE =Selezione pulsantiera Acc.3 pos carico 2

      U     "SL797";
      UN    "M25.6";
      S     "M25.7";
NETWORK
TITLE =Deselezione pulsantiera Acc.3 pos carico 2

      UN    "SL797";
      R     "M25.7";
NETWORK
TITLE =Selezione pulsantiera zona apertura pallet

      U     "PZApertura Pallet";
      UN    "SL680";
      S     "M25.5";
NETWORK
TITLE =Deselezione pulsantiera zona apertura pallet

      UN    "PZApertura Pallet";
      R     "M25.5";
NETWORK
TITLE ======== Consensi Boxing =======



NETWORK
TITLE =CONSENSO MOV + ASSE X

      O     "FC116";
      O     ;
      U     "SL706";
      UN    "FC116";
      UN    "FC117";
      =     "CM+AX";
NETWORK
TITLE =CONSENSO MOV - ASSE X
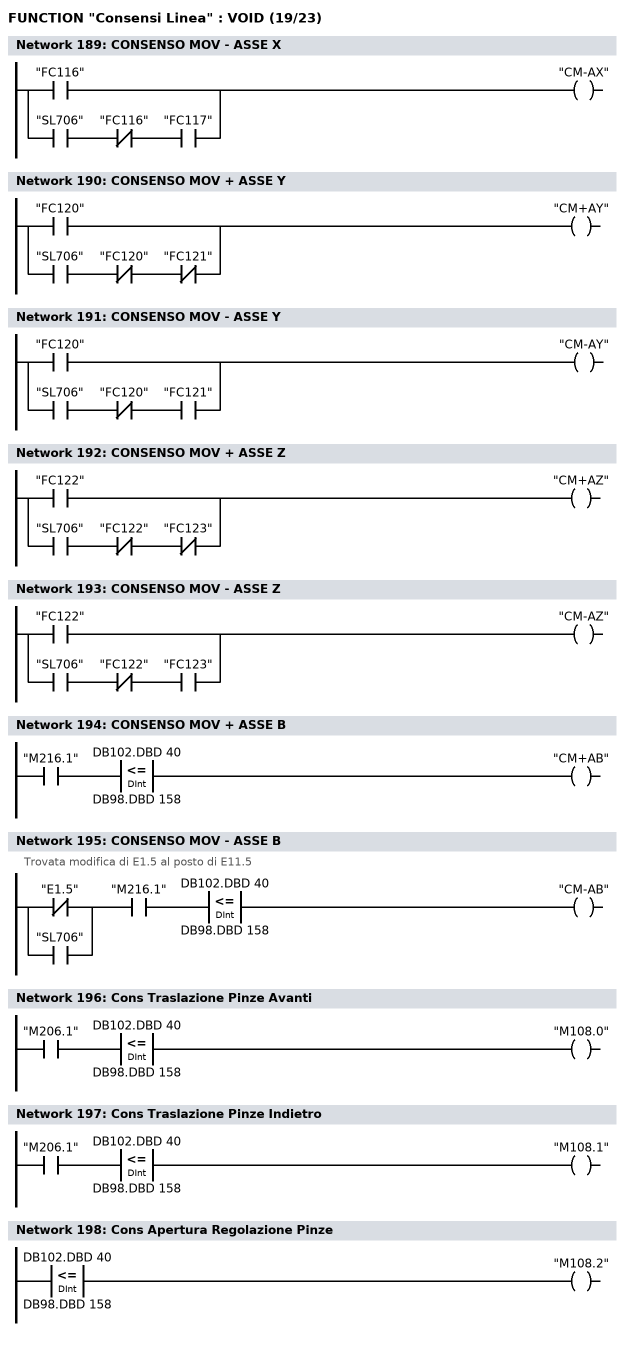
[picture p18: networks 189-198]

      O     "FC116";
      O     ;
      U     "SL706";
      UN    "FC116";
      U     "FC117";
      =     "CM-AX";
NETWORK
TITLE =CONSENSO MOV + ASSE Y

      O     "FC120";
      O     ;
      U     "SL706";
      UN    "FC120";
      UN    "FC121";
      =     "CM+AY";
NETWORK
TITLE =CONSENSO MOV - ASSE Y

      O     "FC120";
      O     ;
      U     "SL706";
      UN    "FC120";
      U     "FC121";
      =     "CM-AY";
NETWORK
TITLE =CONSENSO MOV + ASSE Z

      O     "FC122";
      O     ;
      U     "SL706";
      UN    "FC122";
      UN    "FC123";
      =     "CM+AZ";
NETWORK
TITLE =CONSENSO MOV - ASSE Z

      O     "FC122";
      O     ;
      U     "SL706";
      UN    "FC122";
      U     "FC123";
      =     "CM-AZ";
NETWORK
TITLE =CONSENSO MOV + ASSE B

      U     "M216.1";
      U(    ;
      L     DB102.DBD   40;
      L     DB98.DBD  158;
      <=D   ;
      )     ;
      =     "CM+AB";
NETWORK
TITLE =CONSENSO MOV - ASSE B
//Trovata modifica di E1.5 al posto di E11.5
      U(    ;
      ON    "E1.5";
      O     "SL706";
      )     ;
      U     "M216.1";
      U(    ;
      L     DB102.DBD   40;
      L     DB98.DBD  158;
      <=D   ;
      )     ;
      =     "CM-AB";
NETWORK
TITLE =Cons Traslazione Pinze Avanti

      U     "M206.1";
      U(    ;
      L     DB102.DBD   40;
      L     DB98.DBD  158;
      <=D   ;
      )     ;
      =     "M108.0";
NETWORK
TITLE =Cons Traslazione Pinze Indietro

      U     "M206.1";
      U(    ;
      L     DB102.DBD   40;
      L     DB98.DBD  158;
      <=D   ;
      )     ;
      =     "M108.1";
NETWORK
TITLE =Cons Apertura Regolazione Pinze

      L     DB102.DBD   40;
      L     DB98.DBD  158;
      <=D   ;
      =     "M108.2";
NETWORK
TITLE =Cons Chiusura Regolazione Pinze
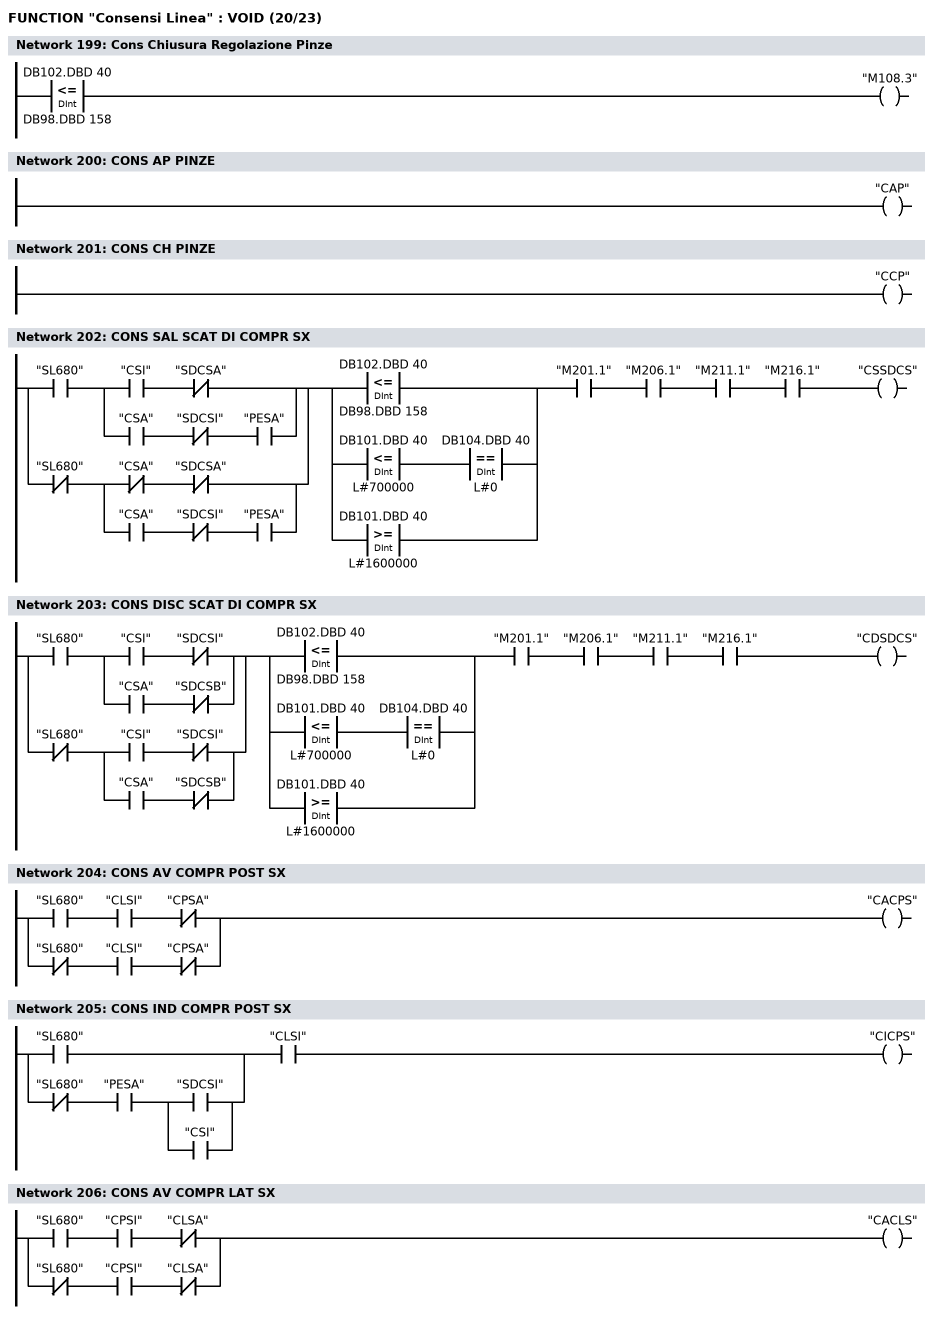
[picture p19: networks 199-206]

      L     DB102.DBD   40;
      L     DB98.DBD  158;
      <=D   ;
      =     "M108.3";
NETWORK
TITLE =CONS AP PINZE

      SET   ;
      =     "CAP";
NETWORK
TITLE =CONS CH PINZE

      SET   ;
      =     "CCP";
NETWORK
TITLE =CONS SAL SCAT DI COMPR SX

      U(    ;
      U     "SL680";
      U(    ;
      U     "CSI";
      UN    "SDCSA";
      O     ;
      U     "CSA";
      UN    "SDCSI";
      U     "PESA";
      )     ;
      O     ;
      UN    "SL680";
      U(    ;
      UN    "CSA";
      UN    "SDCSA";
      O     ;
      U     "CSA";
      UN    "SDCSI";
      U     "PESA";
      )     ;
      )     ;
      U(    ;
      O(    ;
      L     DB102.DBD   40;
      L     DB98.DBD  158;
      <=D   ;
      )     ;
      O     ;
      U(    ;
      L     DB101.DBD   40;
      L     L#700000;
      <=D   ;
      )     ;
      U(    ;
      L     DB104.DBD   40;
      L     L#0;
      ==D   ;
      )     ;
      O(    ;
      L     DB101.DBD   40;
      L     L#1600000;
      >=D   ;
      )     ;
      )     ;
      U     "M201.1";
      U     "M206.1";
      U     "M211.1";
      U     "M216.1";
      =     "CSSDCS";
NETWORK
TITLE =CONS DISC SCAT DI COMPR SX

      U(    ;
      U     "SL680";
      U(    ;
      U     "CSI";
      UN    "SDCSI";
      O     ;
      U     "CSA";
      UN    "SDCSB";
      )     ;
      O     ;
      UN    "SL680";
      U(    ;
      U     "CSI";
      UN    "SDCSI";
      O     ;
      U     "CSA";
      UN    "SDCSB";
      )     ;
      )     ;
      U(    ;
      O(    ;
      L     DB102.DBD   40;
      L     DB98.DBD  158;
      <=D   ;
      )     ;
      O     ;
      U(    ;
      L     DB101.DBD   40;
      L     L#700000;
      <=D   ;
      )     ;
      U(    ;
      L     DB104.DBD   40;
      L     L#0;
      ==D   ;
      )     ;
      O(    ;
      L     DB101.DBD   40;
      L     L#1600000;
      >=D   ;
      )     ;
      )     ;
      U     "M201.1";
      U     "M206.1";
      U     "M211.1";
      U     "M216.1";
      =     "CDSDCS";
NETWORK
TITLE =CONS AV COMPR POST SX

      U     "SL680";
      U     "CLSI";
      UN    "CPSA";
      O     ;
      UN    "SL680";
      U     "CLSI";
      UN    "CPSA";
      =     "CACPS";
NETWORK
TITLE =CONS IND COMPR POST SX

      U(    ;
      O     "SL680";

      O     ;
      UN    "SL680";
      U     "PESA";
      U(    ;
      O     "SDCSI";
      O     "CSI";
      )     ;
      )     ;
      U     "CLSI";
      =     "CICPS";
NETWORK
TITLE =CONS AV COMPR LAT SX

      U     "SL680";
      U     "CPSI";
      UN    "CLSA";
      O     ;
      UN    "SL680";
      U     "CPSI";
      UN    "CLSA";
      =     "CACLS";
NETWORK
TITLE =CONS IND COMPR LAT SX
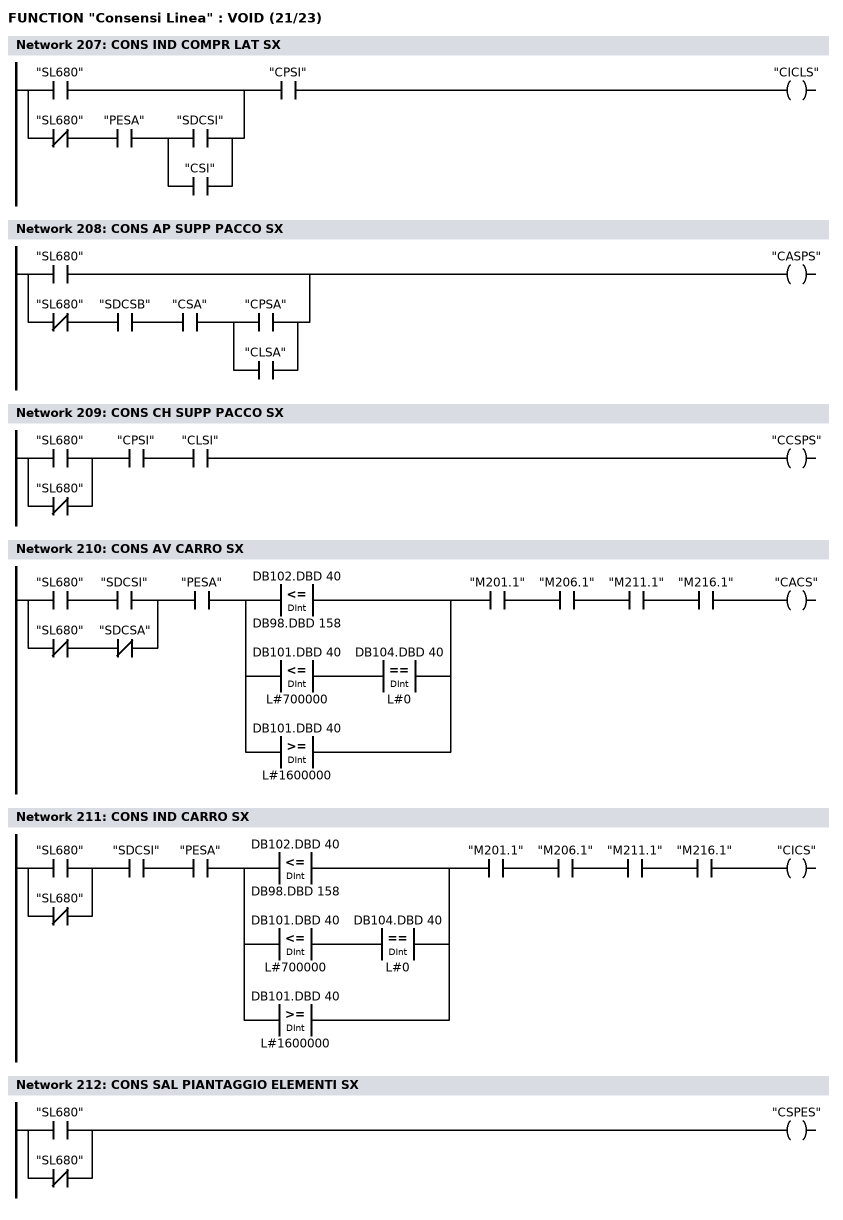
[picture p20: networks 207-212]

      U(    ;
      O     "SL680";
      O     ;
      UN    "SL680";
      U     "PESA";
      U(    ;
      O     "SDCSI";
      O     "CSI";
      )     ;
      )     ;
      U     "CPSI";
      =     "CICLS";
NETWORK
TITLE =CONS AP SUPP PACCO SX

      O     "SL680";
      O     ;
      UN    "SL680";
      U     "SDCSB";
      U     "CSA";
      U(    ;
      O     "CPSA";
      O     "CLSA";
      )     ;
      =     "CASPS";
NETWORK
TITLE =CONS CH SUPP PACCO SX

      U(    ;
      O     "SL680";
      ON    "SL680";
      )     ;
      U     "CPSI";
      U     "CLSI";
      =     "CCSPS";
NETWORK
TITLE =CONS AV CARRO SX

      U(    ;
      U     "SL680";
      U     "SDCSI";
      O     ;
      UN    "SL680";
      UN    "SDCSA";
      )     ;
      U     "PESA";
      U(    ;
      O(    ;
      L     DB102.DBD   40;
      L     DB98.DBD  158;
      <=D   ;
      )     ;
      O     ;
      U(    ;
      L     DB101.DBD   40;
      L     L#700000;
      <=D   ;
      )     ;
      U(    ;
      L     DB104.DBD   40;
      L     L#0;
      ==D   ;
      )     ;
      O(    ;
      L     DB101.DBD   40;
      L     L#1600000;
      >=D   ;
      )     ;
      )     ;
      U     "M201.1";
      U     "M206.1";
      U     "M211.1";
      U     "M216.1";
      =     "CACS";
NETWORK
TITLE =CONS IND CARRO SX

      U(    ;
      O     "SL680";
      ON    "SL680";
      )     ;
      U     "SDCSI";
      U     "PESA";
      U(    ;
      O(    ;
      L     DB102.DBD   40;
      L     DB98.DBD  158;
      <=D   ;
      )     ;
      O     ;
      U(    ;
      L     DB101.DBD   40;
      L     L#700000;
      <=D   ;
      )     ;
      U(    ;
      L     DB104.DBD   40;
      L     L#0;
      ==D   ;
      )     ;
      O(    ;
      L     DB101.DBD   40;
      L     L#1600000;
      >=D   ;
      )     ;
      )     ;
      U     "M201.1";
      U     "M206.1";
      U     "M211.1";
      U     "M216.1";
      =     "CICS";
NETWORK
TITLE =CONS SAL PIANTAGGIO ELEMENTI SX

      O     "SL680";
      ON    "SL680";
      =     "CSPES";
NETWORK
TITLE =CONS DISC PIANTAGGIO ELEMENTI SX
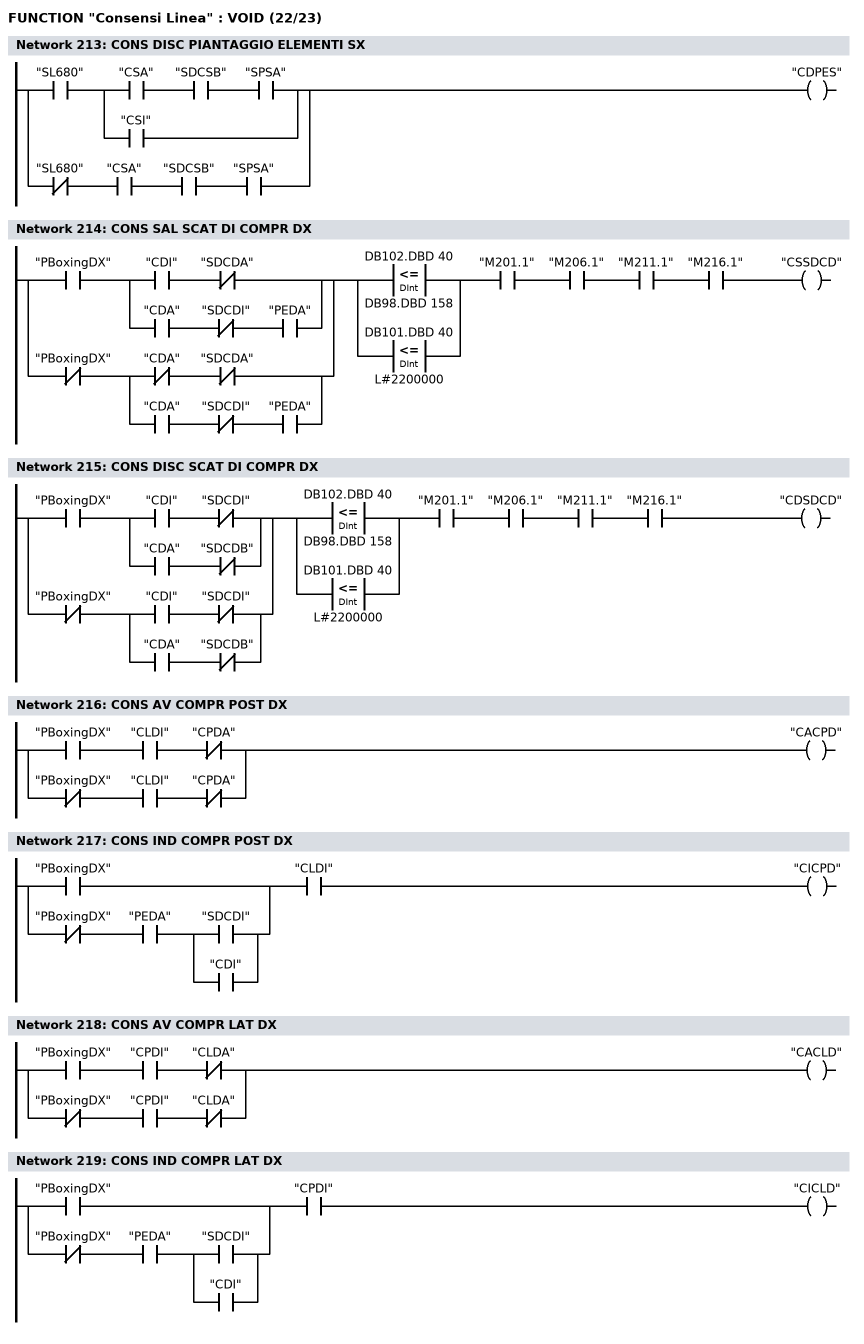
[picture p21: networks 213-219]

      U     "SL680";
      U(    ;
      U     "CSA";
      U     "SDCSB";
      U     "SPSA";
      O     "CSI";
      )     ;
      O     ;
      UN    "SL680";
      U     "CSA";
      U     "SDCSB";
      U     "SPSA";
      =     "CDPES";
NETWORK
TITLE =CONS SAL SCAT DI COMPR DX

      U(    ;
      U     "PBoxingDX";
      U(    ;
      U     "CDI";
      UN    "SDCDA";
      O     ;
      U     "CDA";
      UN    "SDCDI";
      U     "PEDA";
      )     ;
      O     ;
      UN    "PBoxingDX";
      U(    ;
      UN    "CDA";
      UN    "SDCDA";
      O     ;
      U     "CDA";
      UN    "SDCDI";
      U     "PEDA";
      )     ;
      )     ;
      U(    ;
      O(    ;
      L     DB102.DBD   40;
      L     DB98.DBD  158;
      <=D   ;
      )     ;
      O(    ;
      L     DB101.DBD   40;
      L     L#2200000;
      <=D   ;
      )     ;
      )     ;
      U     "M201.1";
      U     "M206.1";
      U     "M211.1";
      U     "M216.1";
      =     "CSSDCD";
NETWORK
TITLE =CONS DISC SCAT DI COMPR DX

      U(    ;
      U     "PBoxingDX";
      U(    ;
      U     "CDI";
      UN    "SDCDI";
      O     ;
      U     "CDA";
      UN    "SDCDB";
      )     ;
      O     ;
      UN    "PBoxingDX";
      U(    ;
      U     "CDI";
      UN    "SDCDI";
      O     ;
      U     "CDA";
      UN    "SDCDB";
      )     ;
      )     ;
      U(    ;
      O(    ;
      L     DB102.DBD   40;
      L     DB98.DBD  158;
      <=D   ;
      )     ;
      O(    ;
      L     DB101.DBD   40;
      L     L#2200000;
      <=D   ;
      )     ;
      )     ;
      U     "M201.1";
      U     "M206.1";
      U     "M211.1";
      U     "M216.1";
      =     "CDSDCD";
NETWORK
TITLE =CONS AV COMPR POST DX

      U     "PBoxingDX";
      U     "CLDI";
      UN    "CPDA";
      O     ;
      UN    "PBoxingDX";
      U     "CLDI";
      UN    "CPDA";
      =     "CACPD";
NETWORK
TITLE =CONS IND COMPR POST DX

      U(    ;
      O     "PBoxingDX";
      O     ;
      UN    "PBoxingDX";
      U     "PEDA";
      U(    ;
      O     "SDCDI";
      O     "CDI";
      )     ;
      )     ;
      U     "CLDI";
      =     "CICPD";
NETWORK
TITLE =CONS AV COMPR LAT DX

      U     "PBoxingDX";
      U     "CPDI";
      UN    "CLDA";
      O     ;
      UN    "PBoxingDX";
      U     "CPDI";
      UN    "CLDA";
      =     "CACLD";
NETWORK
TITLE =CONS IND COMPR LAT DX

      U(    ;
      O     "PBoxingDX";
      O     ;
      UN    "PBoxingDX";
      U     "PEDA";
      U(    ;
      O     "SDCDI";
      O     "CDI";
      )     ;
      )     ;
      U     "CPDI";
      =     "CICLD";
NETWORK
TITLE =CONS AP SUPP PACCO DX
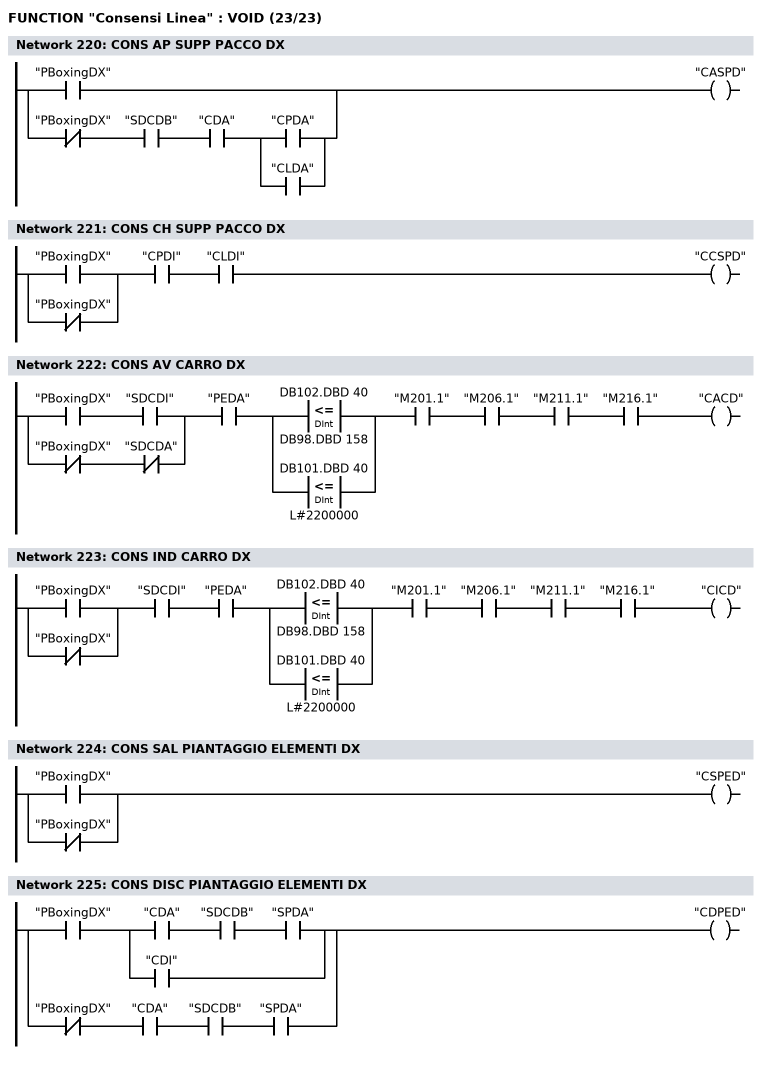
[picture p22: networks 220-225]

      O     "PBoxingDX";
      O     ;
      UN    "PBoxingDX";
      U     "SDCDB";
      U     "CDA";
      U(    ;
      O     "CPDA";
      O     "CLDA";
      )     ;
      =     "CASPD";
NETWORK
TITLE =CONS CH SUPP PACCO DX

      U(    ;
      O     "PBoxingDX";
      ON    "PBoxingDX";
      )     ;
      U     "CPDI";
      U     "CLDI";
      =     "CCSPD";
NETWORK
TITLE =CONS AV CARRO DX

      U(    ;
      U     "PBoxingDX";
      U     "SDCDI";
      O     ;
      UN    "PBoxingDX";
      UN    "SDCDA";
      )     ;
      U     "PEDA";
      U(    ;
      O(    ;
      L     DB102.DBD   40;
      L     DB98.DBD  158;
      <=D   ;
      )     ;
      O(    ;
      L     DB101.DBD   40;
      L     L#2200000;
      <=D   ;
      )     ;
      )     ;
      U     "M201.1";
      U     "M206.1";
      U     "M211.1";
      U     "M216.1";
      =     "CACD";
NETWORK
TITLE =CONS IND CARRO DX

      U(    ;
      O     "PBoxingDX";
      ON    "PBoxingDX";
      )     ;
      U     "SDCDI";
      U     "PEDA";
      U(    ;
      O(    ;
      L     DB102.DBD   40;
      L     DB98.DBD  158;
      <=D   ;
      )     ;
      O(    ;
      L     DB101.DBD   40;
      L     L#2200000;
      <=D   ;
      )     ;
      )     ;
      U     "M201.1";
      U     "M206.1";
      U     "M211.1";
      U     "M216.1";
      =     "CICD";
NETWORK
TITLE =CONS SAL PIANTAGGIO ELEMENTI DX

      O     "PBoxingDX";
      ON    "PBoxingDX";
      =     "CSPED";
NETWORK
TITLE =CONS DISC PIANTAGGIO ELEMENTI DX

      U     "PBoxingDX";
      U(    ;
      U     "CDA";
      U     "SDCDB";
      U     "SPDA";
      O     "CDI";
      )     ;
      O     ;
      UN    "PBoxingDX";
      U     "CDA";
      U     "SDCDB";
      U     "SPDA";
      =     "CDPED";
END_FUNCTION

